(* Logix 5000 AddOnInstructionDefinition export Banner_TL50Pro_Param_v4; software revision 33.00 *)

TYPE Banner_IOL_Port_v4 :   // UDT that has all of the data items necessary to communicate with a specific Port on a IO-Link Master
STRUCT
   Port_Controlled : INT;   // Each bit represents a port on an IO-Link Master. Set to 1 to tell AOI to control that port.
   Port_Activate : INT;   // Each bit represents a port on an IO-Link Master. When ON that port will process any commands in queue.
   Port_Read : INT;   // Each bit represents a port on an IO-Link Master. Used to determine when device AOI has requested a Read command.
   Port_Write : INT;   // Each bit represents a port on an IO-Link Master. Used to determine when device AOI has requested a Write command.
   Port_RW_Complete : INT;   // Each bit represents a port on an IO-Link Master. Tells device AOI that Read or Write request has been completed.
   Port_Device_Read : INT;
   Data_Transfer : SINT[190];   // Array to transfer data from IO-Master to device AOIs.
END_STRUCT
END_TYPE

TYPE Banner_TL50Pro_Basic_SP_v4 :   // Basic parameters for a TL50 Pro segment.
STRUCT
   Animation_Rotational_Direction : SINT;   // 0 = Counter Clockwise, 1 = Clockwise
   Animation_Color_2_Intensity : SINT;   // 0 = High, 1 = Low, 2 = Medium, 3 = Off, 4 = Custom
   Animation_Color_2 : INT;   // 0 = Green, 1 = Red, 2 = Orange, 3 = Amber, 4 = Yellow, 5 = Lime Green, 6 = Spring Green, 7 = Cyan, 8 = Sky Blue, 9 = Blue, 10 = Violet, 11 = Magenta, 12 = Rose, 13 = White, 14 = Custom, 15 = Custom 2
   Animation_Pattern : SINT;   // 0 = Normal, 1 = Strobe, 2 = Three Pulse, 3 = SOS, 4 = Random
   Animation_Speed : SINT;   // 0 = Medium, 1 = Fasr, 2 = Slow, 3 = Custom
   Animation_Color_1_Intensity : SINT;   // 0 = High, 1 = Low, 2 = Medium, 3 = Off, 4 = Custom
   Animation_Color_1 : INT;   // 0 = Green, 1 = Red, 2 = Orange, 3 = Amber, 4 = Yellow, 5 = Lime Green, 6 = Spring Green, 7 = Cyan, 8 = Sky Blue, 9 = Blue, 10 = Violet, 11 = Magenta, 12 = Rose, 13 = White, 14 = Custom, 15 = Custom 2
   Animation : SINT;   // 0 = Off, 1 = Steady, 2 = Flash, 3 = Two Color, 4 = Half/Half, 5 = Half/Half Rotate, 6 = Chase, 7 = Intesnity Sweep
   Basic_Speed : SINT;   // 0 = Medium, 1 = Fast, 2 = Slow, 3 = Custom
   Basic_Color : SINT;   // 0 = Green, 1 = Red, 2 = Orange, 3 = Amber, 4 = Yellow, 5 = Lime Green, 6 = Spring Green, 7 = Cyan, 8 = Sky Blue, 9 = Blue, 10 = Violet, 11 = Magenta, 12 = Rose, 13 = White, 14 = Custom, 15 = Custom 2
END_STRUCT
END_TYPE

TYPE Banner_TL50Pro_RD_v4 :   // UDT that stores the Read Data for a TL50 Pro.
STRUCT
   Master_Cycle_Time : INT;
   Min_Cycle_Time : INT;
   M_Sequence_Capability : INT;
   IO_Link_Version_ID : INT;
   Process_Data_Input_Length : INT;
   Process_Data_Output_Length : INT;
   Combined_Vendor_ID : DINT;   // IO-Link Vendor ID
   Vendor_ID1 : INT;
   Vendor_ID2 : INT;
   Combined_Device_ID : DINT;   // IO-Link Device ID
   Device_ID1 : INT;
   Device_ID2 : INT;
   Device_ID3 : INT;
   Serial_Number : STRING;
END_STRUCT
END_TYPE

TYPE Banner_TL50Pro_v4 :   // All of the parameters for a TL50 Pro.
STRUCT
   Initial_Global_Read : BOOL;   // Determines if all of the IO-Link data has been read into the PLC yet
   Command : INT;   // Value placed in here will activate a read or write to a specifc IO-Link Index
   Read_Data : Banner_TL50Pro_RD_v4;   // Read Only Data
   Write_Data : Banner_TL50Pro_WD_v4;   // Write Data
   Archive_Data : Banner_TL50Pro_WD_v4;   // Archive of the Write Data
   Reset : BOOL;   // Resets AOI. This will force a complete parameter read of the sensor.
END_STRUCT
END_TYPE

TYPE Banner_TL50Pro_WD_v4 :   // UDT that stores the Write Data for a TL50 Pro.
STRUCT
   System_Command : INT;   // See IODD file for list of commands that can be activated via the System Command interface
   Parameter_Access_Lock : SINT;   // Write access to all parameters is prohibited while value is 1. Only this parameter can be adjusted when value is 1.
   Data_Storage_Lock : SINT;   // Automatic data storage is disabled when this value is equal to 1. Read access is not affected.
   Local_Parameterization_Lock : SINT;   // Parameterization via local control elements on device is disabled.
   Local_User_Interface_Lock : SINT;   // Operation of local user interface is disabled.
   Operating_Mode_Selection : SINT;   // 0 = Basic Mode, 1 = Advanced Mode, 2= Run Mode, 3 = Level Mode
   Segment_Basic : Banner_TL50Pro_Basic_SP_v4[11];
   Restrict_to_Gamut : SINT;   // 0 = Off, 1 = On
   Number_of_Segments_for_Scroll_and_Bounce : INT;   // 0 to 10
   Custom_Flash_Rate : INT;   // .5 to 20 Hz (range 5 to 200)
   Custom_Intensity : INT;   // 0 to 100%
   Custom_1_Red : INT;   // 0 to 255. Value of the Red portion of the RGB color value for Custom 1
   Custom_1_Green : INT;   // 0 to 255. Value of the Green portion of the RGB color value for Custom 1.
   Custom_1_Blue : INT;   // 0 to 255. Value of the Blue portion of the RGB color value for Custom 1.
   Custom_2_Red : INT;   // 0 to 255. Value of the Red portion of the RGB color value for Custom 2.
   Custom_2_Green : INT;   // 0 to 255. Value of the Green portion of the RGB color value for Custom 2.
   Custom_2_Blue : INT;   // 0 to 255. Value of the Blue portion of the RGB color value for Custom 2.
   LM_Full_Scale_Value : DINT;
   LM_Base_Color : INT;   // 0 = Green, 1 = Red, 2 = Orange, 3 = Amber, 4 = Yellow, 5 = Lime Green, 6 = Spring Green, 7 = Cyan, 8 = Sky Blue, 9 = Blue, 10 = Violet, 11 = Magenta, 12 = Rose, 13 = White, 14 = Custom, 15 = Custom 2
   LM_Base_Intensity : SINT;   // 0 = High, 1 = Low, 2 = Medium, 3 = Off, 4 = Custom
   LM_Base_State : SINT;   // 0 = Steady, 1 = Flashing
   LM_Threshold_Type : SINT;   // 0 = None, 1 = Low, 2 = High, 3 = High and Low
   LM_Low_Threshold_Value : DINT;
   LM_Low_Threshold_Color : INT;   // 0 = Green, 1 = Red, 2 = Orange, 3 = Amber, 4 = Yellow, 5 = Lime Green, 6 = Spring Green, 7 = Cyan, 8 = Sky Blue, 9 = Blue, 10 = Violet, 11 = Magenta, 12 = Rose, 13 = White, 14 = Custom, 15 = Custom 2
   LM_Low_Threshold_Intensity : SINT;   // 0 = High, 1 = Low, 2 = Medium, 3 = Off, 4 = Custom
   LM_Low_Threshold_State : SINT;   // 0 = Steady, 1 = Flashing
   LM_High_Threshold_Value : DINT;
   LM_High_Threshold_Color : INT;   // 0 = Green, 1 = Red, 2 = Orange, 3 = Amber, 4 = Yellow, 5 = Lime Green, 6 = Spring Green, 7 = Cyan, 8 = Sky Blue, 9 = Blue, 10 = Violet, 11 = Magenta, 12 = Rose, 13 = White, 14 = Custom, 15 = Custom 2
   LM_High_Threshold_Intensity : SINT;   // 0 = High, 1 = Low, 2 = Medium, 3 = Off, 4 = Custom
   LM_High_Threshold_State : SINT;   // 0 = Steady, 1 = Flashing
   LM_Flash_Rate : SINT;   // 0 = Medium, 1 = Fast, 2 = Slow, 3 = Custom
   LM_Dominance : SINT;   // 0 = Dominant, 1 = Non-Dominant
   LM_Subsegment_Style : SINT;   // 0 = Steady, 1 = Flashing, 2 = Analog
   LM_Background_Color : SINT;   // 0 = Green, 1 = Red, 2 = Orange, 3 = Amber, 4 = Yellow, 5 = Lime Green, 6 = Spring Green, 7 = Cyan, 8 = Sky Blue, 9 = Blue, 10 = Violet, 11 = Magenta, 12 = Rose, 13 = White, 14 = Custom, 15 = Custom 2
   LM_Background_Intensity : SINT;   // 0 = High, 1 = Low, 2 = Medium, 3 = Off, 4 = Custom
   LM_Orientation : SINT;   // 0 = Steady, 1 = Flashing
END_STRUCT
END_TYPE

ADD_ON_INSTRUCTION Banner_TL50Pro_Param_v4   (* revision 4.1, vendor Banner Engineering *)
// AOI to read and write parameter data to an IO-Link TL50 Pro.
VAR_IN_OUT
   TL50_Pro : Banner_TL50Pro_v4; {required}
   Port_Data : Banner_IOL_Port_v4; {required}
END_VAR
VAR_INPUT
   Port : INT; {required}   // Port Number that device is plugged into.
END_VAR
VAR
   Local_Control : DINT; {access None}
   Global_Read_Command_Value : INT; {access None}
   Global_Write_Command_Value : INT; {access None}
   Command_Being_Processed : BOOL; {access None}
   Update_Archive : BOOL; {access None}
   Index_Write_Inprocess : DINT; {access None}
   Index_Write_Control : DINT; {access None}
   Inprocess_Index : DINT; {access None}
   Index_R_Segment : DINT; {access None}
   BS_Index : DINT; {access None}
   Index_W_Segment : DINT; {access None}
   SB_W_Index : DINT; {access None}
   Index_Segment_Read : DINT; {access None}
END_VAR

ROUTINE Logic   (* ladder *)
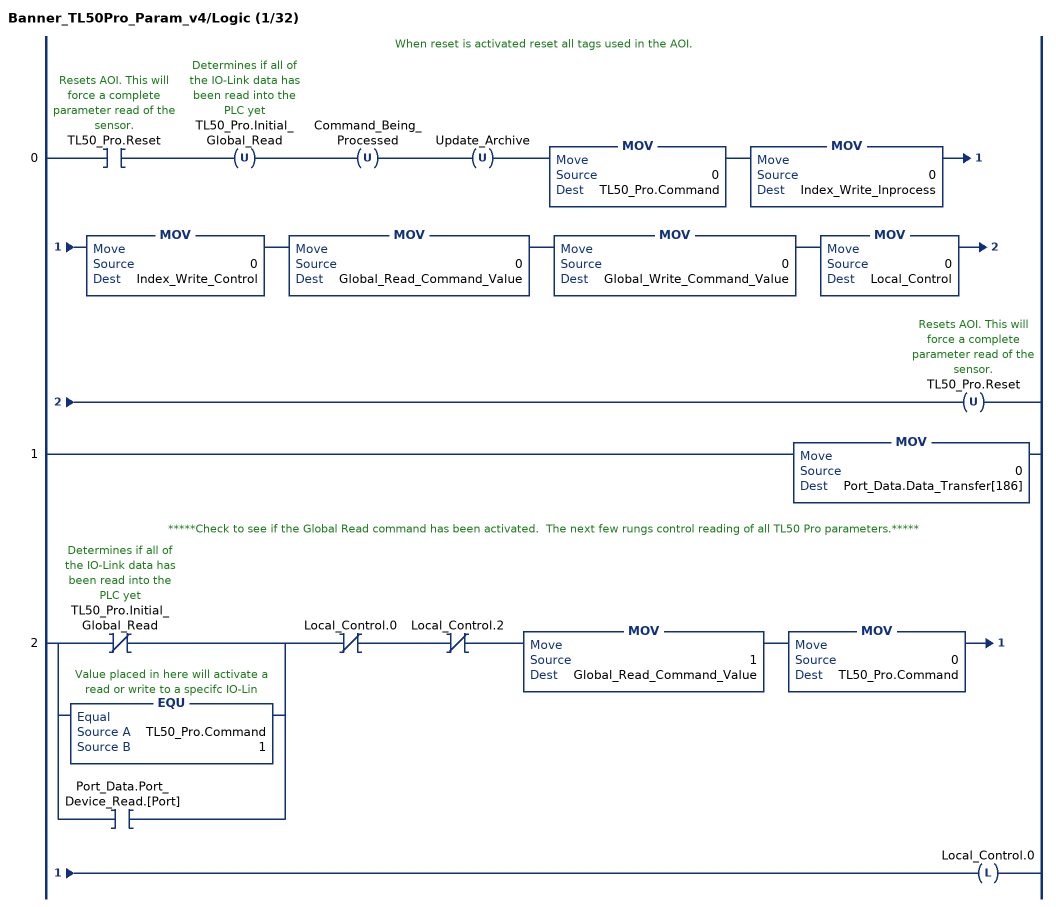
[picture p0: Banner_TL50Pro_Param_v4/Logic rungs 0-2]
   // When reset is activated reset all tags used in the AOI.
   0: XIC(TL50_Pro.Reset)OTU(TL50_Pro.Initial_Global_Read)OTU(Command_Being_Processed)OTU(Update_Archive)MOV(0,TL50_Pro.Command)MOV(0,Index_Write_Inprocess)MOV(0,Index_Write_Control)MOV(0,Global_Read_Command_Value)MOV(0,Global_Write_Command_Value)MOV(0,Local_Control)OTU(TL50_Pro.Reset);
   1: MOV(0,Port_Data.Data_Transfer[186]);
   // *****Check to see if the Global Read command has been activated.  The next few rungs control reading of all TL50 Pro parameters.*****
   2: [XIO(TL50_Pro.Initial_Global_Read) ,EQU(TL50_Pro.Command,1) ,XIC(Port_Data.Port_Device_Read.[Port]) ]XIO(Local_Control.0)XIO(Local_Control.2)MOV(1,Global_Read_Command_Value)MOV(0,TL50_Pro.Command)OTL(Local_Control.0);
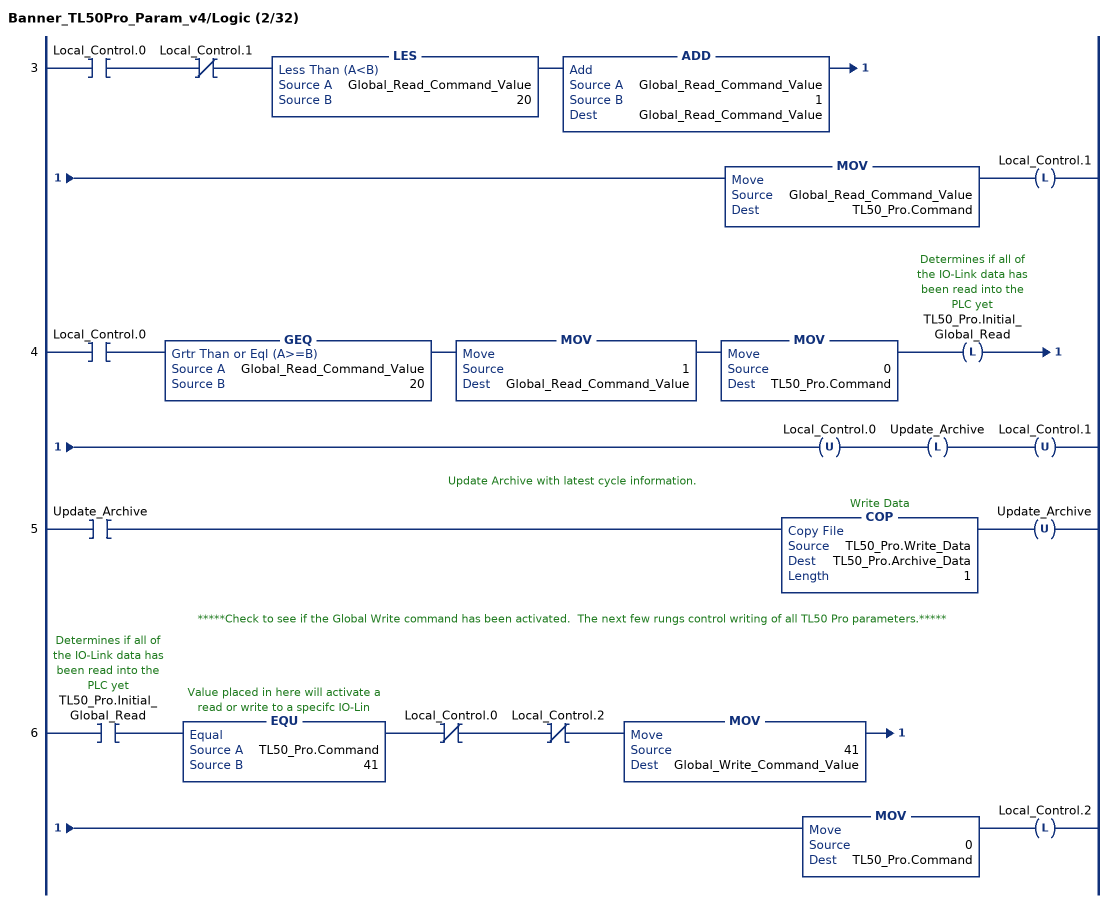
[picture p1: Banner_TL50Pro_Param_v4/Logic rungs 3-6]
   3: XIC(Local_Control.0)XIO(Local_Control.1)LES(Global_Read_Command_Value,20)ADD(Global_Read_Command_Value,1,Global_Read_Command_Value)MOV(Global_Read_Command_Value,TL50_Pro.Command)OTL(Local_Control.1);
   4: XIC(Local_Control.0)GEQ(Global_Read_Command_Value,20)MOV(1,Global_Read_Command_Value)MOV(0,TL50_Pro.Command)OTL(TL50_Pro.Initial_Global_Read)OTU(Local_Control.0)OTL(Update_Archive)OTU(Local_Control.1);
   // Update Archive with latest cycle information.
   5: XIC(Update_Archive)COP(TL50_Pro.Write_Data,TL50_Pro.Archive_Data,1)OTU(Update_Archive);
   // *****Check to see if the Global Write command has been activated.  The next few rungs control writing of all TL50 Pro parameters.*****
   6: XIC(TL50_Pro.Initial_Global_Read)EQU(TL50_Pro.Command,41)XIO(Local_Control.0)XIO(Local_Control.2)MOV(41,Global_Write_Command_Value)MOV(0,TL50_Pro.Command)OTL(Local_Control.2);
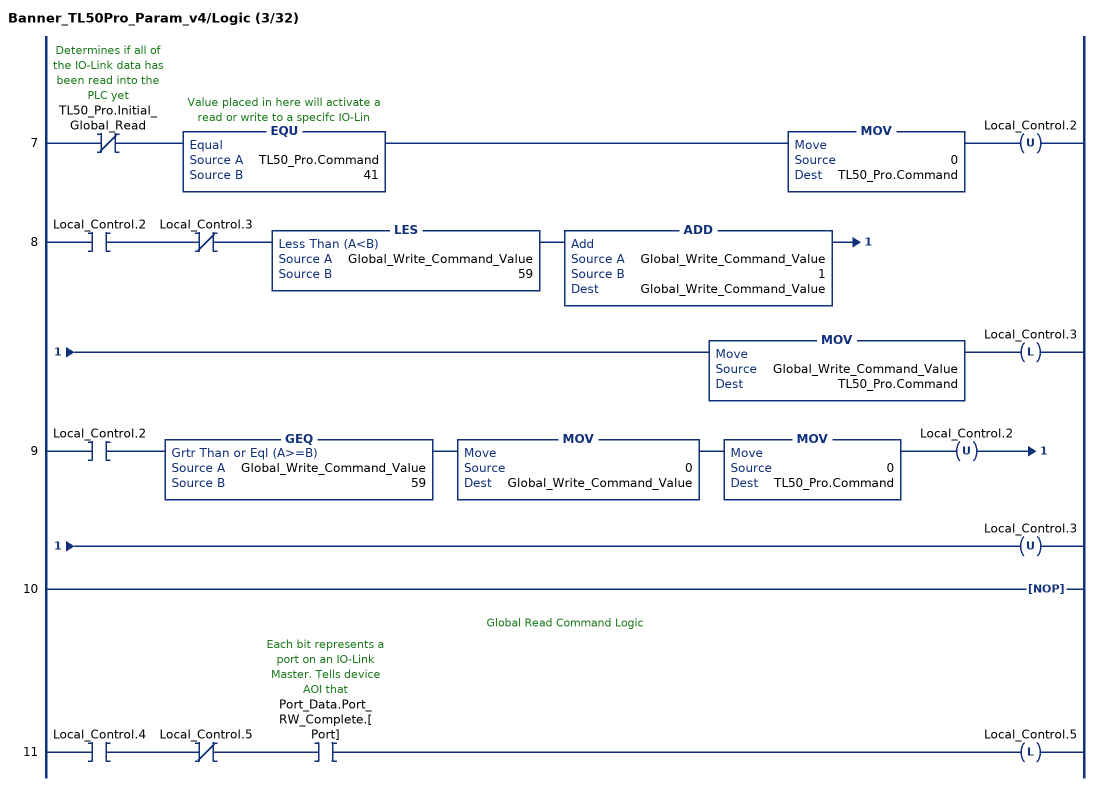
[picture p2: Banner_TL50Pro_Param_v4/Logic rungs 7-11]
   7: XIO(TL50_Pro.Initial_Global_Read)EQU(TL50_Pro.Command,41)MOV(0,TL50_Pro.Command)OTU(Local_Control.2);
   8: XIC(Local_Control.2)XIO(Local_Control.3)LES(Global_Write_Command_Value,59)ADD(Global_Write_Command_Value,1,Global_Write_Command_Value)MOV(Global_Write_Command_Value,TL50_Pro.Command)OTL(Local_Control.3);
   9: XIC(Local_Control.2)GEQ(Global_Write_Command_Value,59)MOV(0,Global_Write_Command_Value)MOV(0,TL50_Pro.Command)OTU(Local_Control.2)OTU(Local_Control.3);
   10: NOP();
   // Global Read Command Logic
   11: XIC(Local_Control.4)XIO(Local_Control.5)XIC(Port_Data.Port_RW_Complete.[Port])OTL(Local_Control.5);
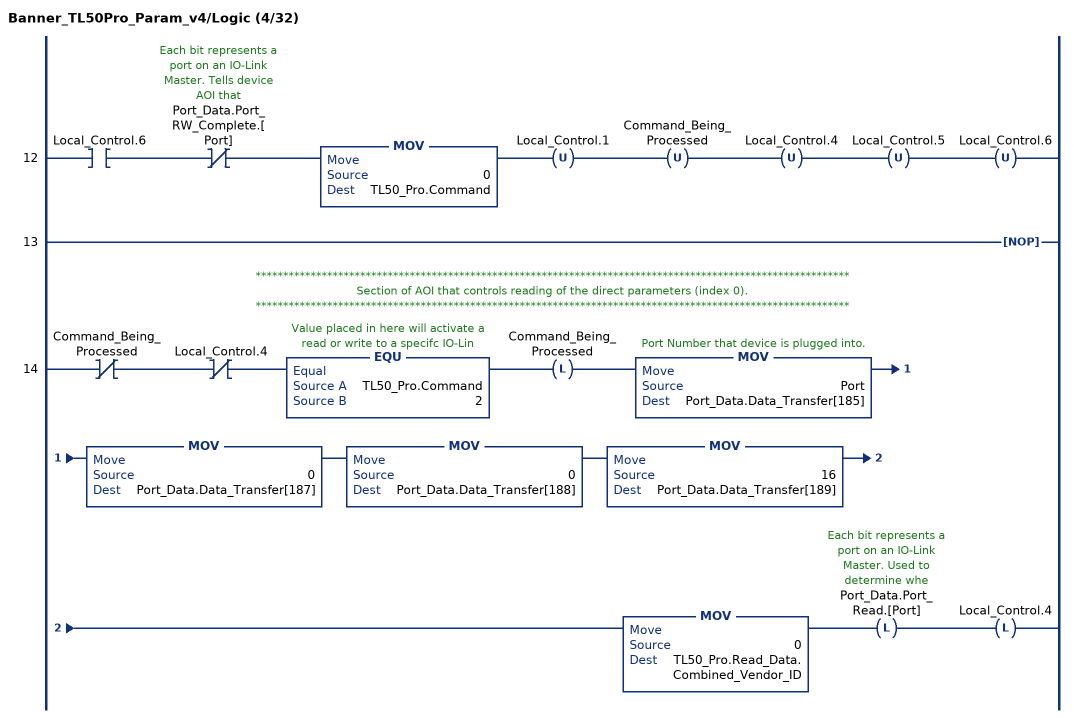
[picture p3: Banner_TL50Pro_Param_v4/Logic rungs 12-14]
   12: XIC(Local_Control.6)XIO(Port_Data.Port_RW_Complete.[Port])MOV(0,TL50_Pro.Command)OTU(Local_Control.1)OTU(Command_Being_Processed)OTU(Local_Control.4)OTU(Local_Control.5)OTU(Local_Control.6);
   13: NOP();
   // ************************************************************************************************************
   // Section of AOI that controls reading of the direct parameters (index 0).
   // ************************************************************************************************************
   14: XIO(Command_Being_Processed)XIO(Local_Control.4)EQU(TL50_Pro.Command,2)OTL(Command_Being_Processed)MOV(Port,Port_Data.Data_Transfer[185])MOV(0,Port_Data.Data_Transfer[187])MOV(0,Port_Data.Data_Transfer[188])MOV(16,Port_Data.Data_Transfer[189])MOV(0,TL50_Pro.Read_Data.Combined_Vendor_ID)OTL(Port_Data.Port_Read.[Port])OTL(Local_Control.4);
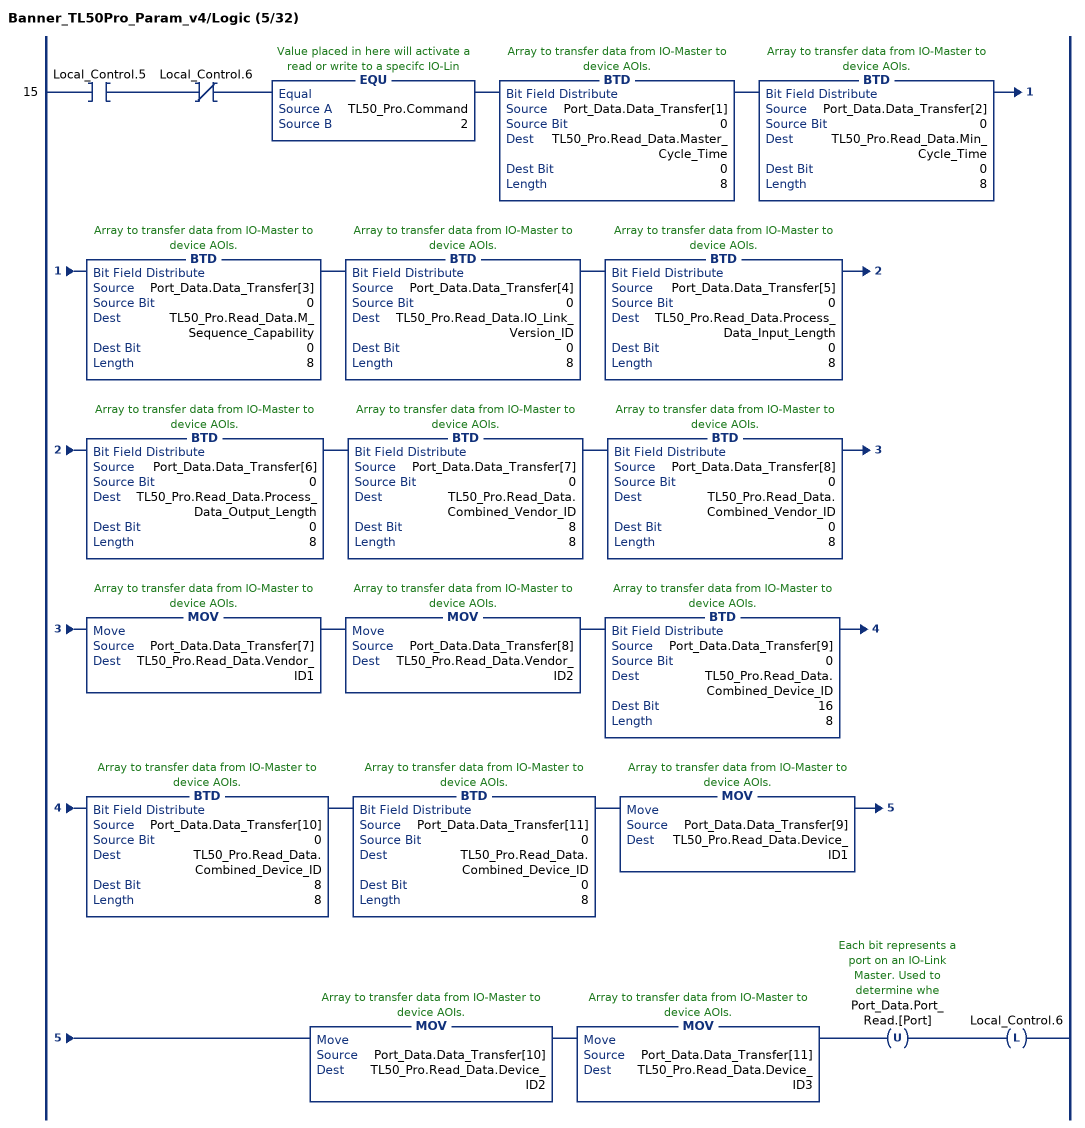
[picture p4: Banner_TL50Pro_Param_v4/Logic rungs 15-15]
   15: XIC(Local_Control.5)XIO(Local_Control.6)EQU(TL50_Pro.Command,2)BTD(Port_Data.Data_Transfer[1],0,TL50_Pro.Read_Data.Master_Cycle_Time,0,8)BTD(Port_Data.Data_Transfer[2],0,TL50_Pro.Read_Data.Min_Cycle_Time,0,8)BTD(Port_Data.Data_Transfer[3],0,TL50_Pro.Read_Data.M_Sequence_Capability,0,8)BTD(Port_Data.Data_Transfer[4],0,TL50_Pro.Read_Data.IO_Link_Version_ID,0,8)BTD(Port_Data.Data_Transfer[5],0,TL50_Pro.Read_Data.Process_Data_Input_Length,0,8)BTD(Port_Data.Data_Transfer[6],0,TL50_Pro.Read_Data.Process_Data_Output_Length,0,8)BTD(Port_Data.Data_Transfer[7],0,TL50_Pro.Read_Data.Combined_Vendor_ID,8,8)BTD(Port_Data.Data_Transfer[8],0,TL50_Pro.Read_Data.Combined_Vendor_ID,0,8)MOV(Port_Data.Data_Transfer[7],TL50_Pro.Read_Data.Vendor_ID1)MOV(Port_Data.Data_Transfer[8],TL50_Pro.Read_Data.Vendor_ID2)BTD(Port_Data.Data_Transfer[9],0,TL50_Pro.Read_Data.Combined_Device_ID,16,8)BTD(Port_Data.Data_Transfer[10],0,TL50_Pro.Read_Data.Combined_Device_ID,8,8)BTD(Port_Data.Data_Transfer[11],0,TL50_Pro.Read_Data.Combined_Device_ID,0,8)MOV(Port_Data.Data_Transfer[9],TL50_Pro.Read_Data.Device_ID1)MOV(Port_Data.Data_Transfer[10],TL50_Pro.Read_Data.Device_ID2)MOV(Port_Data.Data_Transfer[11],TL50_Pro.Read_Data.Device_ID3)OTU(Port_Data.Port_Read.[Port])OTL(Local_Control.6);
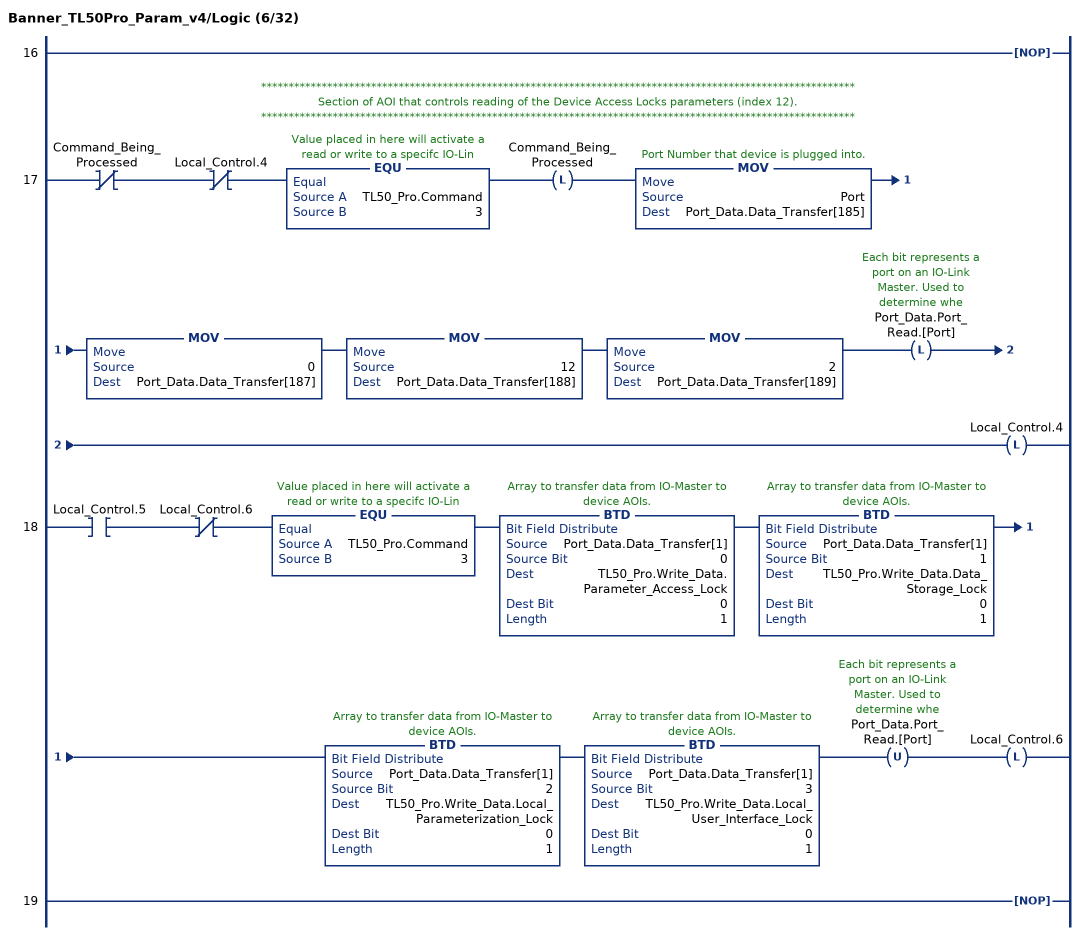
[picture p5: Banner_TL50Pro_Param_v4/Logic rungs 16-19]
   16: NOP();
   // ************************************************************************************************************
   // Section of AOI that controls reading of the Device Access Locks parameters (index 12).
   // ************************************************************************************************************
   17: XIO(Command_Being_Processed)XIO(Local_Control.4)EQU(TL50_Pro.Command,3)OTL(Command_Being_Processed)MOV(Port,Port_Data.Data_Transfer[185])MOV(0,Port_Data.Data_Transfer[187])MOV(12,Port_Data.Data_Transfer[188])MOV(2,Port_Data.Data_Transfer[189])OTL(Port_Data.Port_Read.[Port])OTL(Local_Control.4);
   18: XIC(Local_Control.5)XIO(Local_Control.6)EQU(TL50_Pro.Command,3)BTD(Port_Data.Data_Transfer[1],0,TL50_Pro.Write_Data.Parameter_Access_Lock,0,1)BTD(Port_Data.Data_Transfer[1],1,TL50_Pro.Write_Data.Data_Storage_Lock,0,1)BTD(Port_Data.Data_Transfer[1],2,TL50_Pro.Write_Data.Local_Parameterization_Lock,0,1)BTD(Port_Data.Data_Transfer[1],3,TL50_Pro.Write_Data.Local_User_Interface_Lock,0,1)OTU(Port_Data.Port_Read.[Port])OTL(Local_Control.6);
   19: NOP();
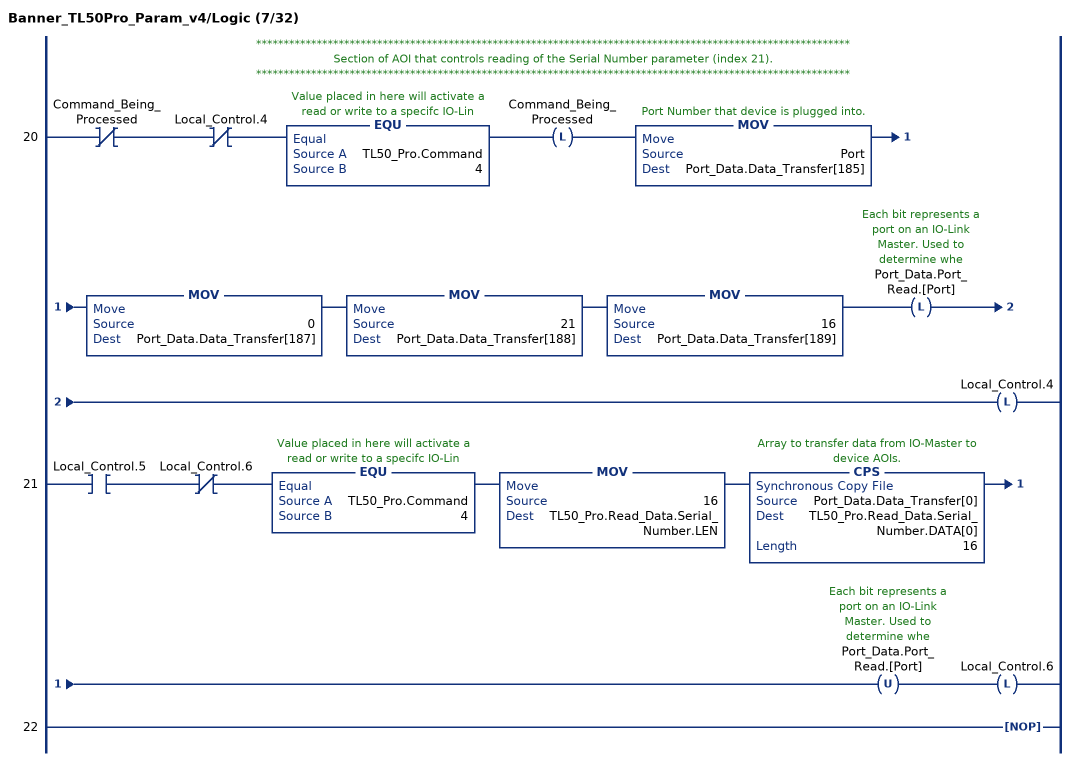
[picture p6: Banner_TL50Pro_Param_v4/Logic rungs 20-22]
   // ************************************************************************************************************
   // Section of AOI that controls reading of the Serial Number parameter (index 21).
   // ************************************************************************************************************
   20: XIO(Command_Being_Processed)XIO(Local_Control.4)EQU(TL50_Pro.Command,4)OTL(Command_Being_Processed)MOV(Port,Port_Data.Data_Transfer[185])MOV(0,Port_Data.Data_Transfer[187])MOV(21,Port_Data.Data_Transfer[188])MOV(16,Port_Data.Data_Transfer[189])OTL(Port_Data.Port_Read.[Port])OTL(Local_Control.4);
   21: XIC(Local_Control.5)XIO(Local_Control.6)EQU(TL50_Pro.Command,4)MOV(16,TL50_Pro.Read_Data.Serial_Number.LEN)CPS(Port_Data.Data_Transfer[0],TL50_Pro.Read_Data.Serial_Number.DATA[0],16)OTU(Port_Data.Port_Read.[Port])OTL(Local_Control.6);
   22: NOP();
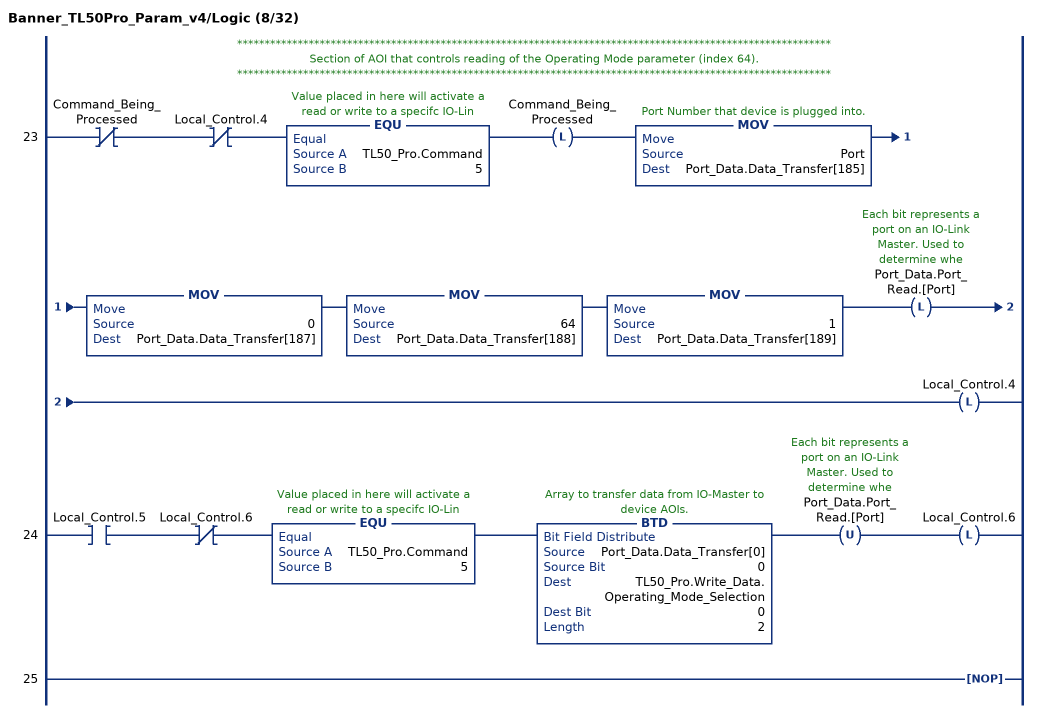
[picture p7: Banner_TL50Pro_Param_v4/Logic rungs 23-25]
   // ************************************************************************************************************
   // Section of AOI that controls reading of the Operating Mode parameter (index 64).
   // ************************************************************************************************************
   23: XIO(Command_Being_Processed)XIO(Local_Control.4)EQU(TL50_Pro.Command,5)OTL(Command_Being_Processed)MOV(Port,Port_Data.Data_Transfer[185])MOV(0,Port_Data.Data_Transfer[187])MOV(64,Port_Data.Data_Transfer[188])MOV(1,Port_Data.Data_Transfer[189])OTL(Port_Data.Port_Read.[Port])OTL(Local_Control.4);
   24: XIC(Local_Control.5)XIO(Local_Control.6)EQU(TL50_Pro.Command,5)BTD(Port_Data.Data_Transfer[0],0,TL50_Pro.Write_Data.Operating_Mode_Selection,0,2)OTU(Port_Data.Port_Read.[Port])OTL(Local_Control.6);
   25: NOP();
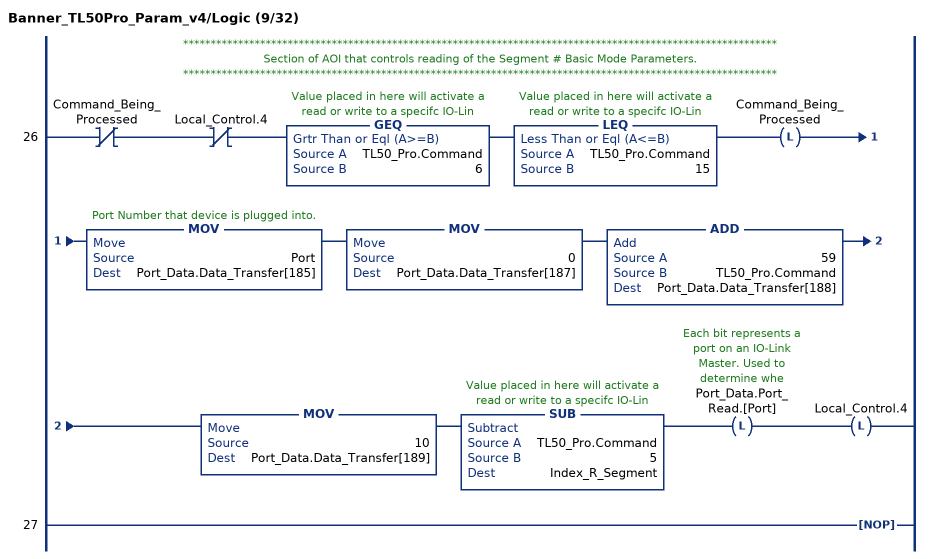
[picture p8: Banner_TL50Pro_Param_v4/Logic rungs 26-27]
   // ************************************************************************************************************
   // Section of AOI that controls reading of the Segment # Basic Mode Parameters.
   // ************************************************************************************************************
   26: XIO(Command_Being_Processed)XIO(Local_Control.4)GEQ(TL50_Pro.Command,6)LEQ(TL50_Pro.Command,15)OTL(Command_Being_Processed)MOV(Port,Port_Data.Data_Transfer[185])MOV(0,Port_Data.Data_Transfer[187])ADD(59,TL50_Pro.Command,Port_Data.Data_Transfer[188])MOV(10,Port_Data.Data_Transfer[189])SUB(TL50_Pro.Command,5,Index_R_Segment)OTL(Port_Data.Port_Read.[Port])OTL(Local_Control.4);
   27: NOP();
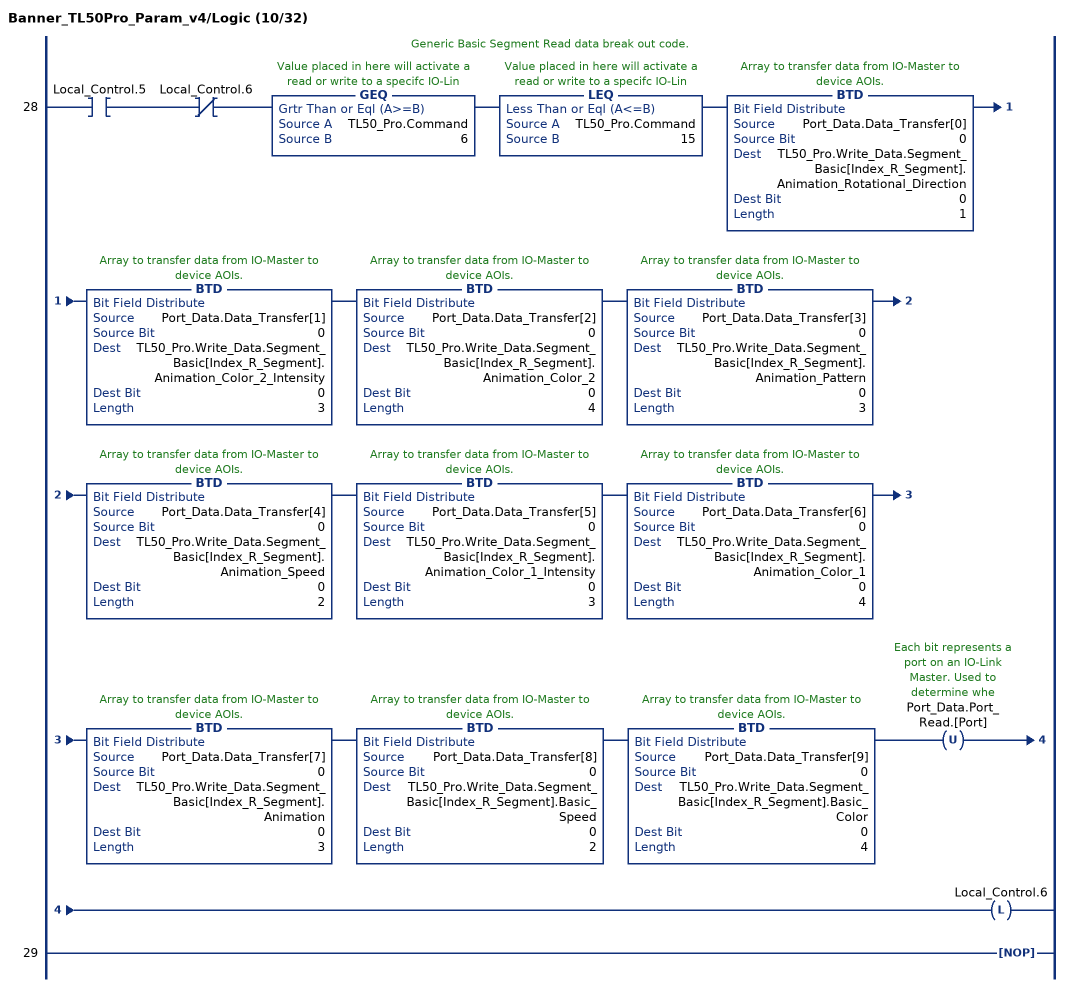
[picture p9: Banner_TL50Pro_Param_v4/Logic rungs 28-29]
   // Generic Basic Segment Read data break out code.
   28: XIC(Local_Control.5)XIO(Local_Control.6)GEQ(TL50_Pro.Command,6)LEQ(TL50_Pro.Command,15)BTD(Port_Data.Data_Transfer[0],0,TL50_Pro.Write_Data.Segment_Basic[Index_R_Segment].Animation_Rotational_Direction,0,1)BTD(Port_Data.Data_Transfer[1],0,TL50_Pro.Write_Data.Segment_Basic[Index_R_Segment].Animation_Color_2_Intensity,0,3)BTD(Port_Data.Data_Transfer[2],0,TL50_Pro.Write_Data.Segment_Basic[Index_R_Segment].Animation_Color_2,0,4)BTD(Port_Data.Data_Transfer[3],0,TL50_Pro.Write_Data.Segment_Basic[Index_R_Segment].Animation_Pattern,0,3)BTD(Port_Data.Data_Transfer[4],0,TL50_Pro.Write_Data.Segment_Basic[Index_R_Segment].Animation_Speed,0,2)BTD(Port_Data.Data_Transfer[5],0,TL50_Pro.Write_Data.Segment_Basic[Index_R_Segment].Animation_Color_1_Intensity,0,3)BTD(Port_Data.Data_Transfer[6],0,TL50_Pro.Write_Data.Segment_Basic[Index_R_Segment].Animation_Color_1,0,4)BTD(Port_Data.Data_Transfer[7],0,TL50_Pro.Write_Data.Segment_Basic[Index_R_Segment].Animation,0,3)BTD(Port_Data.Data_Transfer[8],0,TL50_Pro.Write_Data.Segment_Basic[Index_R_Segment].Basic_Speed,0,2)BTD(Port_Data.Data_Transfer[9],0,TL50_Pro.Write_Data.Segment_Basic[Index_R_Segment].Basic_Color,0,4)OTU(Port_Data.Port_Read.[Port])OTL(Local_Control.6);
   29: NOP();
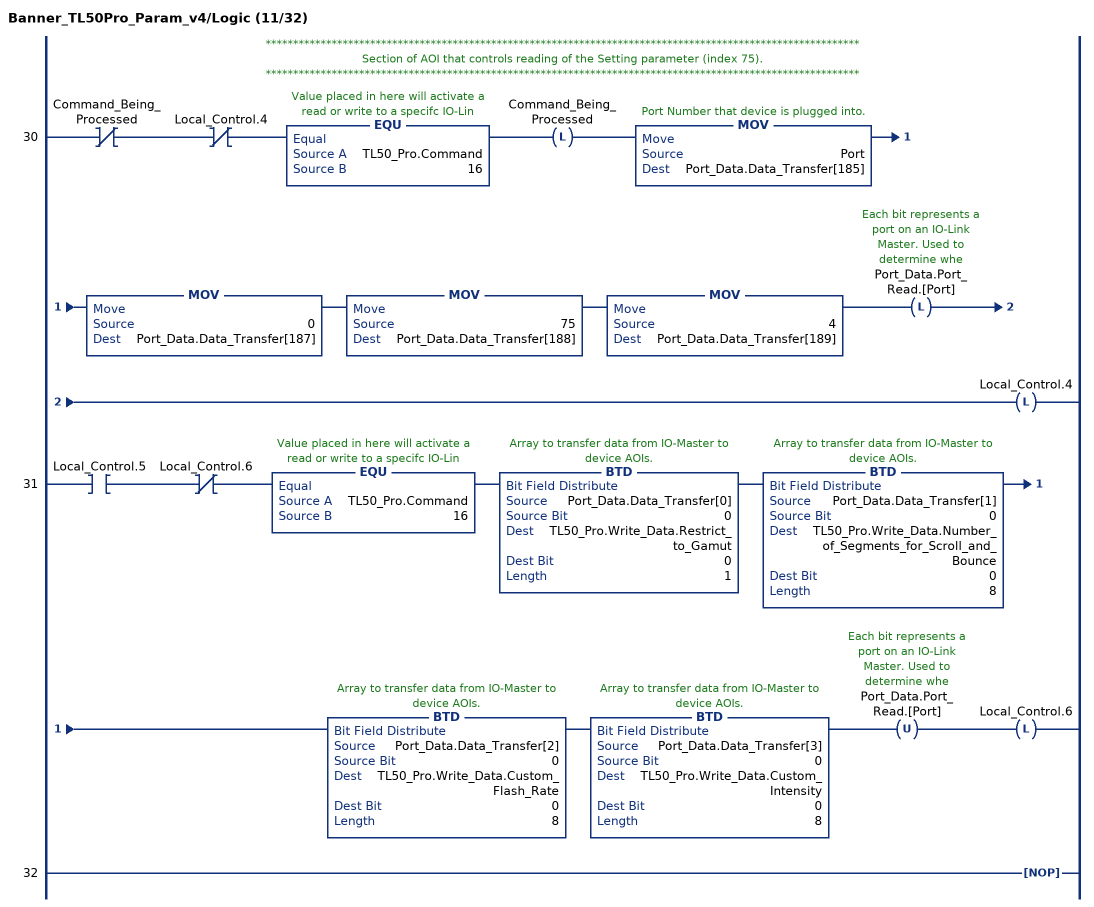
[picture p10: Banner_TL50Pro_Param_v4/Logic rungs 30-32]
   // ************************************************************************************************************
   // Section of AOI that controls reading of the Setting parameter (index 75).
   // ************************************************************************************************************
   30: XIO(Command_Being_Processed)XIO(Local_Control.4)EQU(TL50_Pro.Command,16)OTL(Command_Being_Processed)MOV(Port,Port_Data.Data_Transfer[185])MOV(0,Port_Data.Data_Transfer[187])MOV(75,Port_Data.Data_Transfer[188])MOV(4,Port_Data.Data_Transfer[189])OTL(Port_Data.Port_Read.[Port])OTL(Local_Control.4);
   31: XIC(Local_Control.5)XIO(Local_Control.6)EQU(TL50_Pro.Command,16)BTD(Port_Data.Data_Transfer[0],0,TL50_Pro.Write_Data.Restrict_to_Gamut,0,1)BTD(Port_Data.Data_Transfer[1],0,TL50_Pro.Write_Data.Number_of_Segments_for_Scroll_and_Bounce,0,8)BTD(Port_Data.Data_Transfer[2],0,TL50_Pro.Write_Data.Custom_Flash_Rate,0,8)BTD(Port_Data.Data_Transfer[3],0,TL50_Pro.Write_Data.Custom_Intensity,0,8)OTU(Port_Data.Port_Read.[Port])OTL(Local_Control.6);
   32: NOP();
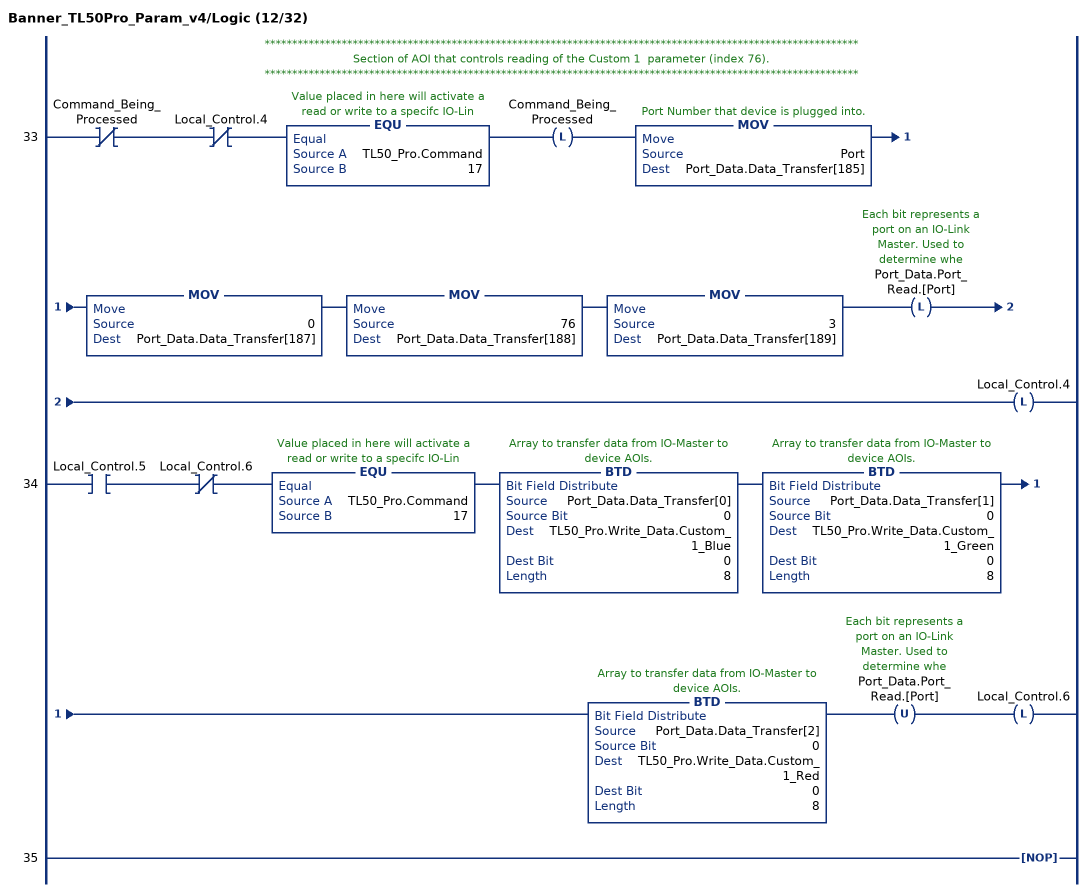
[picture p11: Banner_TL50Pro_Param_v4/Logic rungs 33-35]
   // ************************************************************************************************************
   // Section of AOI that controls reading of the Custom 1  parameter (index 76).
   // ************************************************************************************************************
   33: XIO(Command_Being_Processed)XIO(Local_Control.4)EQU(TL50_Pro.Command,17)OTL(Command_Being_Processed)MOV(Port,Port_Data.Data_Transfer[185])MOV(0,Port_Data.Data_Transfer[187])MOV(76,Port_Data.Data_Transfer[188])MOV(3,Port_Data.Data_Transfer[189])OTL(Port_Data.Port_Read.[Port])OTL(Local_Control.4);
   34: XIC(Local_Control.5)XIO(Local_Control.6)EQU(TL50_Pro.Command,17)BTD(Port_Data.Data_Transfer[0],0,TL50_Pro.Write_Data.Custom_1_Blue,0,8)BTD(Port_Data.Data_Transfer[1],0,TL50_Pro.Write_Data.Custom_1_Green,0,8)BTD(Port_Data.Data_Transfer[2],0,TL50_Pro.Write_Data.Custom_1_Red,0,8)OTU(Port_Data.Port_Read.[Port])OTL(Local_Control.6);
   35: NOP();
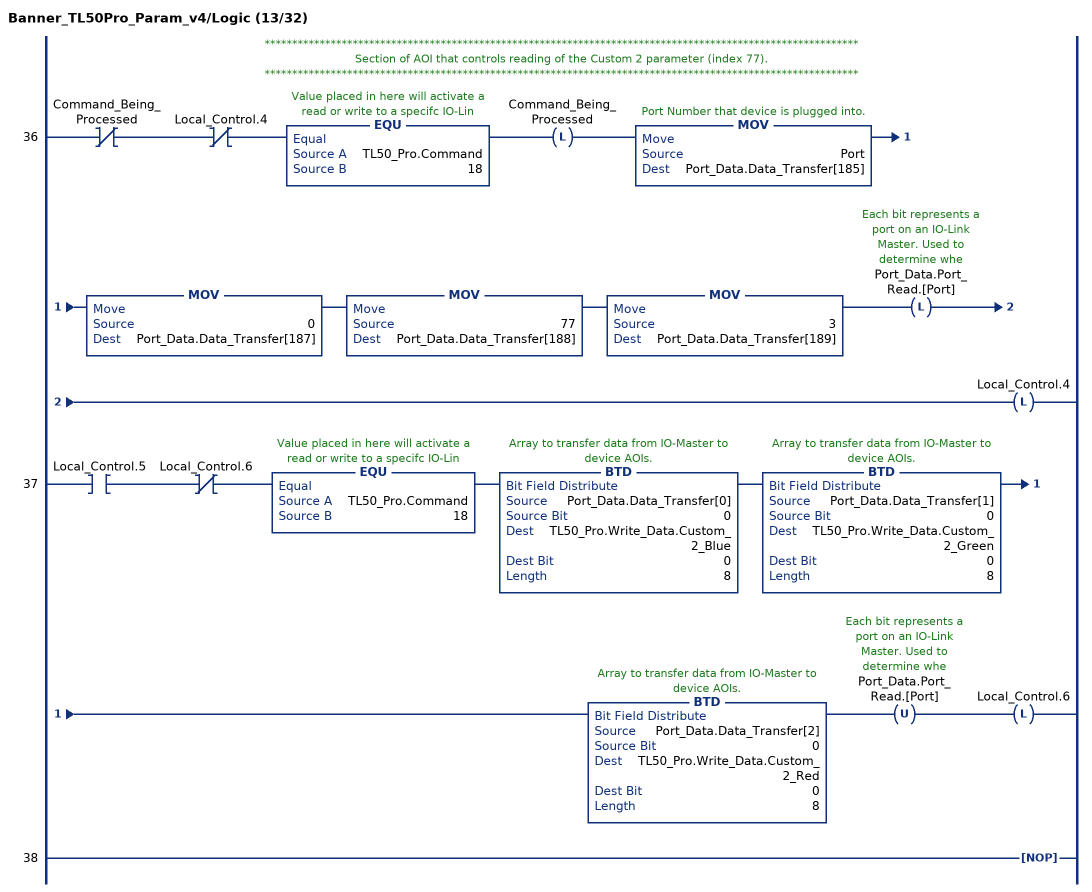
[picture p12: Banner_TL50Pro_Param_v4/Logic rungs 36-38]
   // ************************************************************************************************************
   // Section of AOI that controls reading of the Custom 2 parameter (index 77).
   // ************************************************************************************************************
   36: XIO(Command_Being_Processed)XIO(Local_Control.4)EQU(TL50_Pro.Command,18)OTL(Command_Being_Processed)MOV(Port,Port_Data.Data_Transfer[185])MOV(0,Port_Data.Data_Transfer[187])MOV(77,Port_Data.Data_Transfer[188])MOV(3,Port_Data.Data_Transfer[189])OTL(Port_Data.Port_Read.[Port])OTL(Local_Control.4);
   37: XIC(Local_Control.5)XIO(Local_Control.6)EQU(TL50_Pro.Command,18)BTD(Port_Data.Data_Transfer[0],0,TL50_Pro.Write_Data.Custom_2_Blue,0,8)BTD(Port_Data.Data_Transfer[1],0,TL50_Pro.Write_Data.Custom_2_Green,0,8)BTD(Port_Data.Data_Transfer[2],0,TL50_Pro.Write_Data.Custom_2_Red,0,8)OTU(Port_Data.Port_Read.[Port])OTL(Local_Control.6);
   38: NOP();
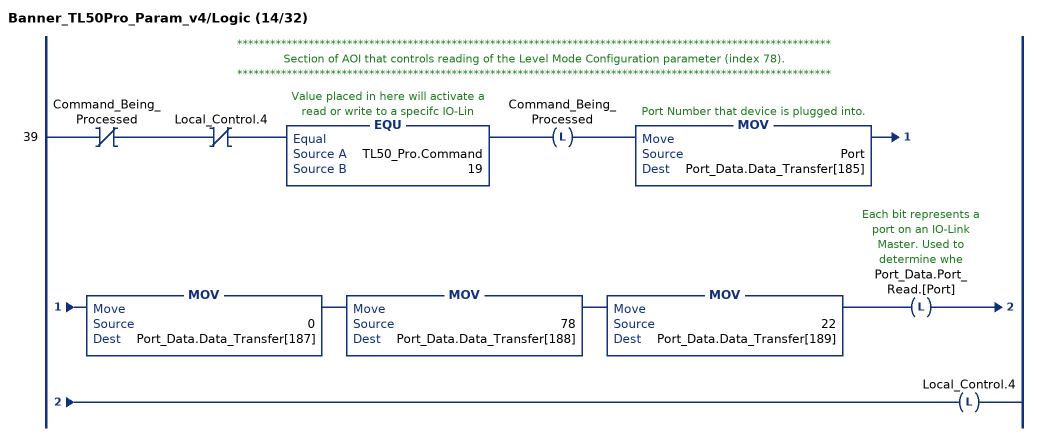
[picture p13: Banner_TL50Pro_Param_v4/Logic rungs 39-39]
   // ************************************************************************************************************
   // Section of AOI that controls reading of the Level Mode Configuration parameter (index 78).
   // ************************************************************************************************************
   39: XIO(Command_Being_Processed)XIO(Local_Control.4)EQU(TL50_Pro.Command,19)OTL(Command_Being_Processed)MOV(Port,Port_Data.Data_Transfer[185])MOV(0,Port_Data.Data_Transfer[187])MOV(78,Port_Data.Data_Transfer[188])MOV(22,Port_Data.Data_Transfer[189])OTL(Port_Data.Port_Read.[Port])OTL(Local_Control.4);
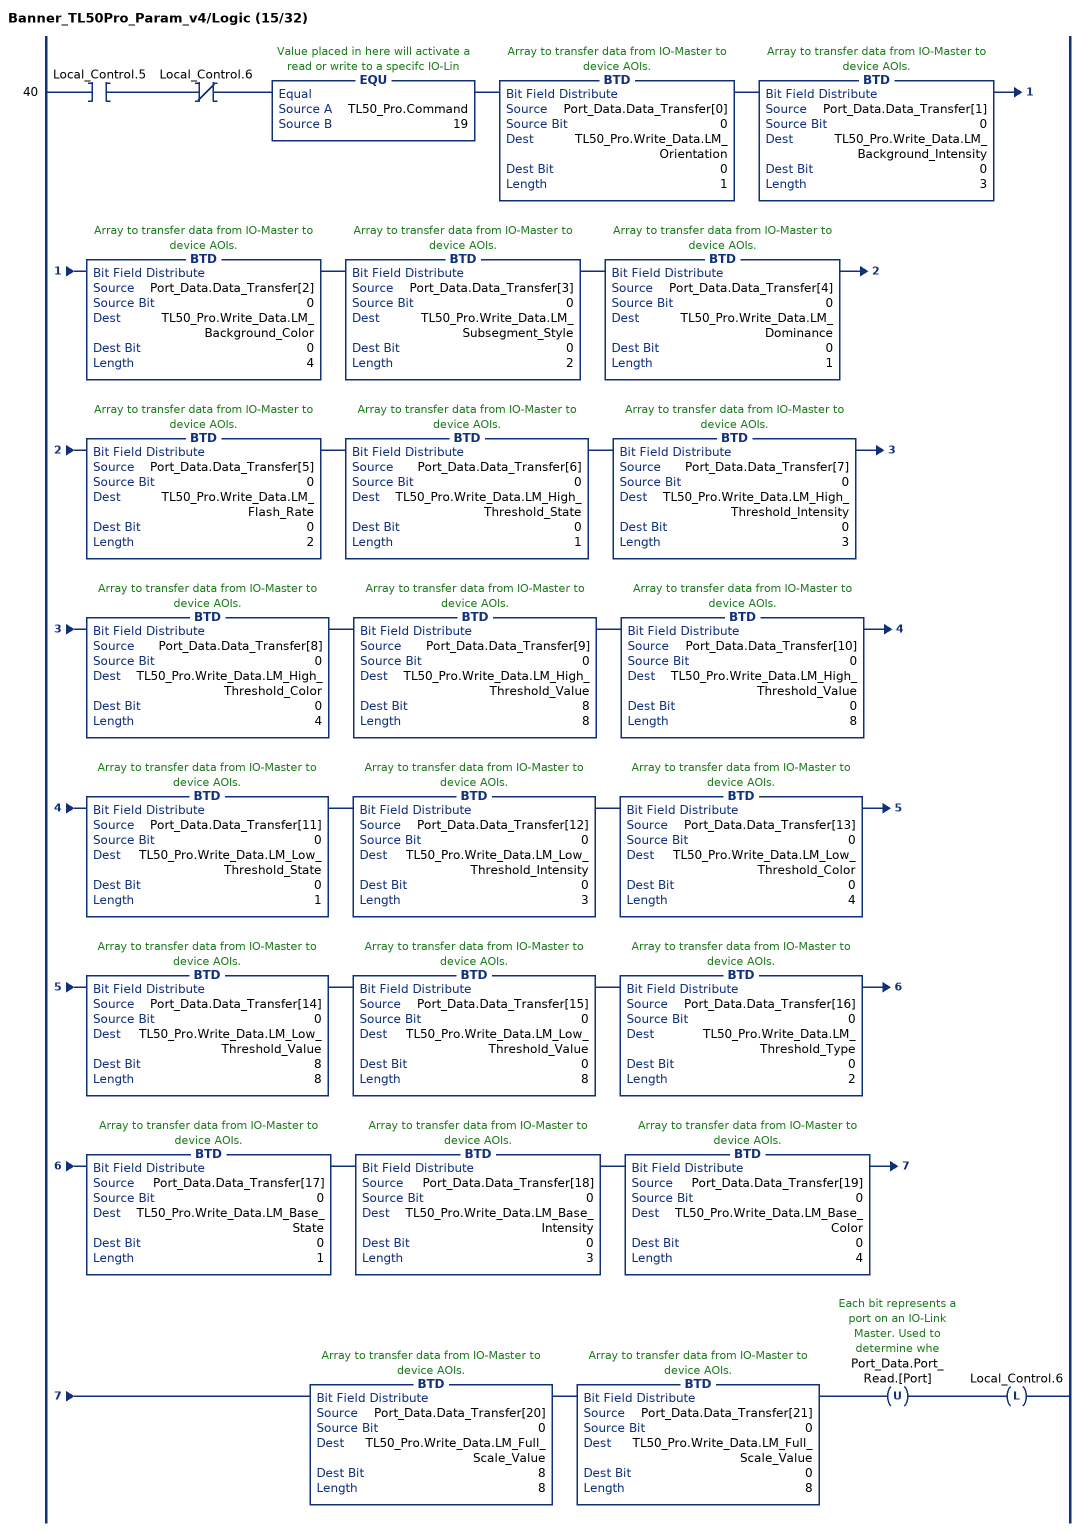
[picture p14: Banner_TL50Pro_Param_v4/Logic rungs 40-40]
   40: XIC(Local_Control.5)XIO(Local_Control.6)EQU(TL50_Pro.Command,19)BTD(Port_Data.Data_Transfer[0],0,TL50_Pro.Write_Data.LM_Orientation,0,1)BTD(Port_Data.Data_Transfer[1],0,TL50_Pro.Write_Data.LM_Background_Intensity,0,3)BTD(Port_Data.Data_Transfer[2],0,TL50_Pro.Write_Data.LM_Background_Color,0,4)BTD(Port_Data.Data_Transfer[3],0,TL50_Pro.Write_Data.LM_Subsegment_Style,0,2)BTD(Port_Data.Data_Transfer[4],0,TL50_Pro.Write_Data.LM_Dominance,0,1)BTD(Port_Data.Data_Transfer[5],0,TL50_Pro.Write_Data.LM_Flash_Rate,0,2)BTD(Port_Data.Data_Transfer[6],0,TL50_Pro.Write_Data.LM_High_Threshold_State,0,1)BTD(Port_Data.Data_Transfer[7],0,TL50_Pro.Write_Data.LM_High_Threshold_Intensity,0,3)BTD(Port_Data.Data_Transfer[8],0,TL50_Pro.Write_Data.LM_High_Threshold_Color,0,4)BTD(Port_Data.Data_Transfer[9],0,TL50_Pro.Write_Data.LM_High_Threshold_Value,8,8)BTD(Port_Data.Data_Transfer[10],0,TL50_Pro.Write_Data.LM_High_Threshold_Value,0,8)BTD(Port_Data.Data_Transfer[11],0,TL50_Pro.Write_Data.LM_Low_Threshold_State,0,1)BTD(Port_Data.Data_Transfer[12],0,TL50_Pro.Write_Data.LM_Low_Threshold_Intensity,0,3)BTD(Port_Data.Data_Transfer[13],0,TL50_Pro.Write_Data.LM_Low_Threshold_Color,0,4)BTD(Port_Data.Data_Transfer[14],0,TL50_Pro.Write_Data.LM_Low_Threshold_Value,8,8)BTD(Port_Data.Data_Transfer[15],0,TL50_Pro.Write_Data.LM_Low_Threshold_Value,0,8)BTD(Port_Data.Data_Transfer[16],0,TL50_Pro.Write_Data.LM_Threshold_Type,0,2)BTD(Port_Data.Data_Transfer[17],0,TL50_Pro.Write_Data.LM_Base_State,0,1)BTD(Port_Data.Data_Transfer[18],0,TL50_Pro.Write_Data.LM_Base_Intensity,0,3)BTD(Port_Data.Data_Transfer[19],0,TL50_Pro.Write_Data.LM_Base_Color,0,4)BTD(Port_Data.Data_Transfer[20],0,TL50_Pro.Write_Data.LM_Full_Scale_Value,8,8)BTD(Port_Data.Data_Transfer[21],0,TL50_Pro.Write_Data.LM_Full_Scale_Value,0,8)OTU(Port_Data.Port_Read.[Port])OTL(Local_Control.6);
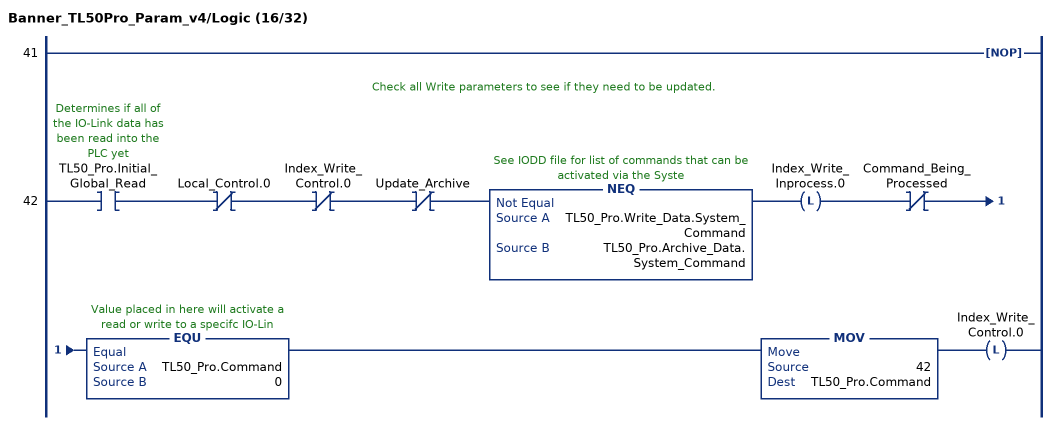
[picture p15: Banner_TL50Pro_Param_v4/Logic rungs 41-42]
   41: NOP();
   // Check all Write parameters to see if they need to be updated.
   42: XIC(TL50_Pro.Initial_Global_Read)XIO(Local_Control.0)XIO(Index_Write_Control.0)XIO(Update_Archive)NEQ(TL50_Pro.Write_Data.System_Command,TL50_Pro.Archive_Data.System_Command)OTL(Index_Write_Inprocess.0)XIO(Command_Being_Processed)EQU(TL50_Pro.Command,0)MOV(42,TL50_Pro.Command)OTL(Index_Write_Control.0);
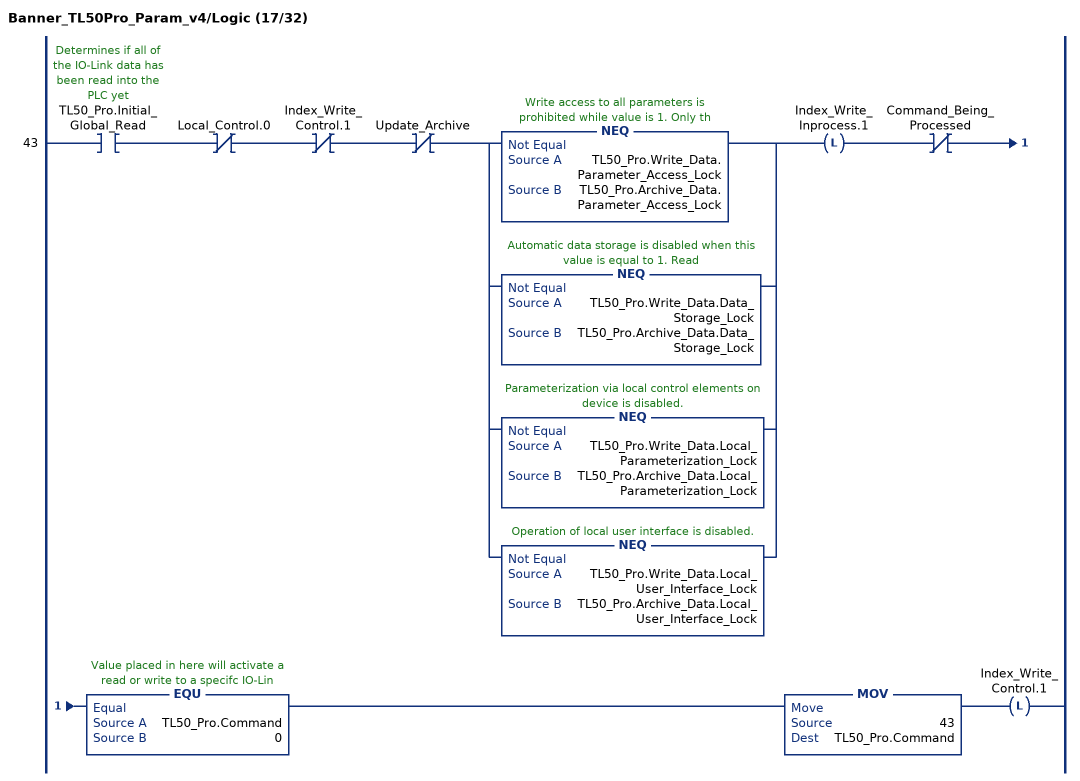
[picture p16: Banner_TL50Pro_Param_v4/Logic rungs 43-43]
   43: XIC(TL50_Pro.Initial_Global_Read)XIO(Local_Control.0)XIO(Index_Write_Control.1)XIO(Update_Archive)[NEQ(TL50_Pro.Write_Data.Parameter_Access_Lock,TL50_Pro.Archive_Data.Parameter_Access_Lock) ,NEQ(TL50_Pro.Write_Data.Data_Storage_Lock,TL50_Pro.Archive_Data.Data_Storage_Lock) ,NEQ(TL50_Pro.Write_Data.Local_Parameterization_Lock,TL50_Pro.Archive_Data.Local_Parameterization_Lock) ,NEQ(TL50_Pro.Write_Data.Local_User_Interface_Lock,TL50_Pro.Archive_Data.Local_User_Interface_Lock) ]OTL(Index_Write_Inprocess.1)XIO(Command_Being_Processed)EQU(TL50_Pro.Command,0)MOV(43,TL50_Pro.Command)OTL(Index_Write_Control.1);
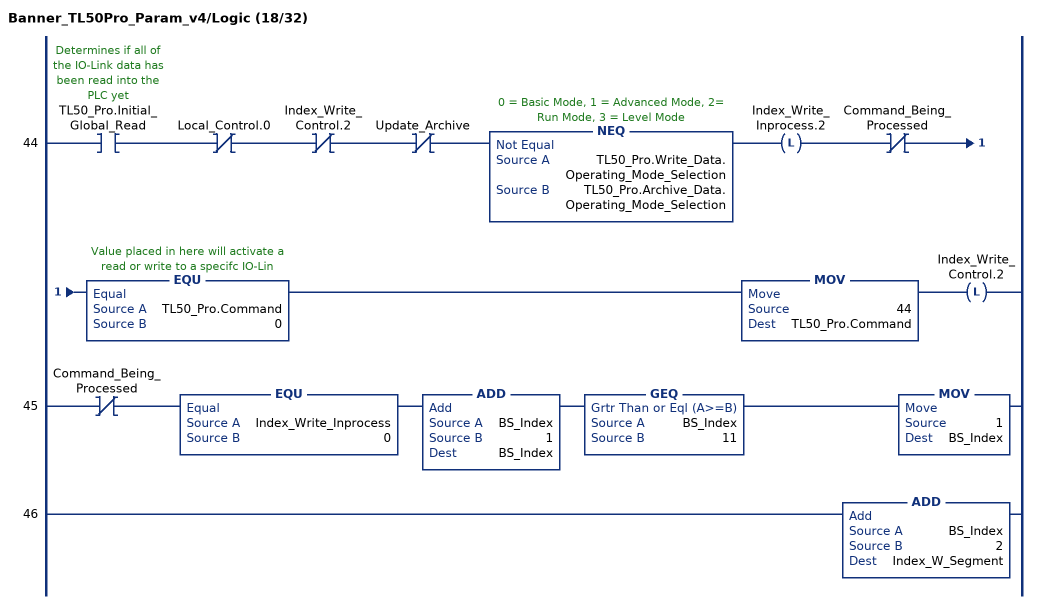
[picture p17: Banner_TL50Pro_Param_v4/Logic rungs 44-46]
   44: XIC(TL50_Pro.Initial_Global_Read)XIO(Local_Control.0)XIO(Index_Write_Control.2)XIO(Update_Archive)NEQ(TL50_Pro.Write_Data.Operating_Mode_Selection,TL50_Pro.Archive_Data.Operating_Mode_Selection)OTL(Index_Write_Inprocess.2)XIO(Command_Being_Processed)EQU(TL50_Pro.Command,0)MOV(44,TL50_Pro.Command)OTL(Index_Write_Control.2);
   45: XIO(Command_Being_Processed)EQU(Index_Write_Inprocess,0)ADD(BS_Index,1,BS_Index)GEQ(BS_Index,11)MOV(1,BS_Index);
   46: ADD(BS_Index,2,Index_W_Segment);
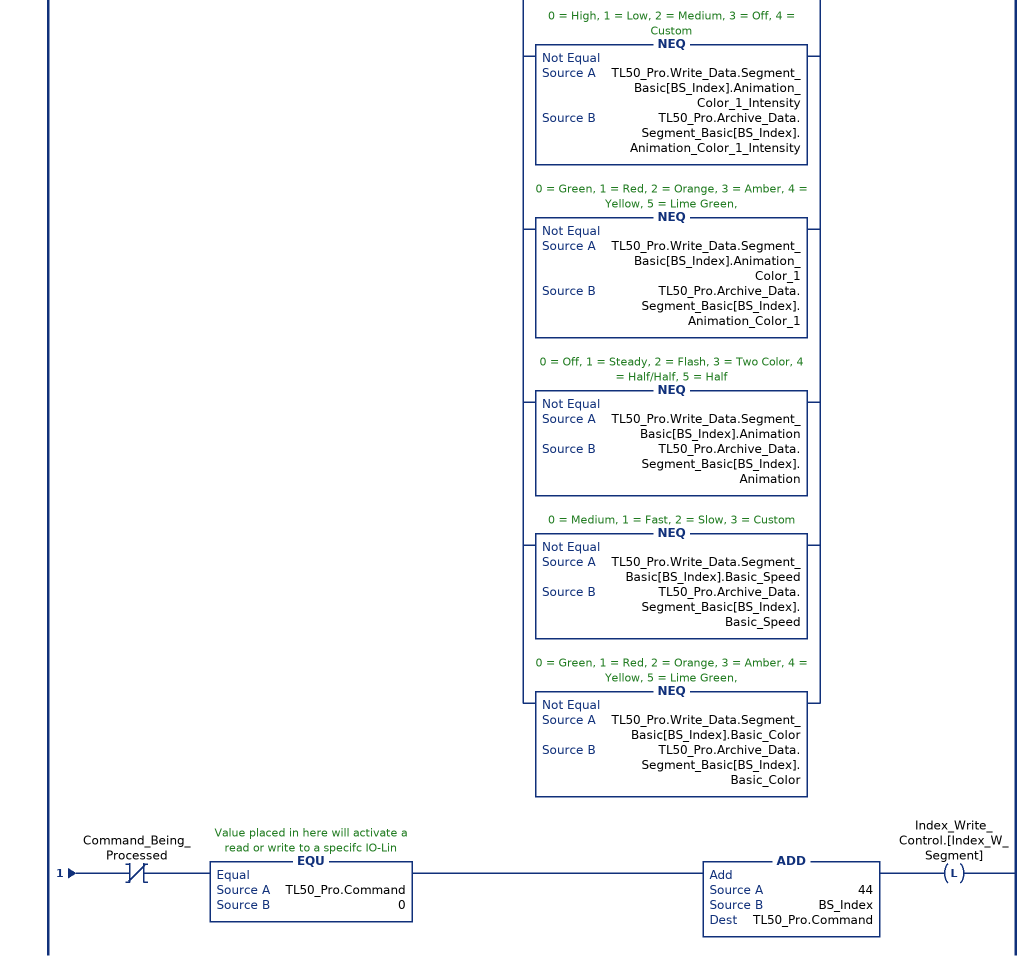
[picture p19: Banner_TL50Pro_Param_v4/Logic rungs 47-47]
   47: XIC(TL50_Pro.Initial_Global_Read)XIO(Local_Control.0)XIO(Index_Write_Control.[Index_W_Segment])XIO(Update_Archive)[NEQ(TL50_Pro.Write_Data.Segment_Basic[BS_Index].Animation_Rotational_Direction,TL50_Pro.Archive_Data.Segment_Basic[BS_Index].Animation_Rotational_Direction) ,NEQ(TL50_Pro.Write_Data.Segment_Basic[BS_Index].Animation_Color_2_Intensity,TL50_Pro.Archive_Data.Segment_Basic[BS_Index].Animation_Color_2_Intensity) ,NEQ(TL50_Pro.Write_Data.Segment_Basic[BS_Index].Animation_Color_2,TL50_Pro.Archive_Data.Segment_Basic[BS_Index].Animation_Color_2) ,NEQ(TL50_Pro.Write_Data.Segment_Basic[BS_Index].Animation_Pattern,TL50_Pro.Archive_Data.Segment_Basic[BS_Index].Animation_Pattern) ,NEQ(TL50_Pro.Write_Data.Segment_Basic[BS_Index].Animation_Speed,TL50_Pro.Archive_Data.Segment_Basic[BS_Index].Animation_Speed) ,NEQ(TL50_Pro.Write_Data.Segment_Basic[BS_Index].Animation_Color_1_Intensity,TL50_Pro.Archive_Data.Segment_Basic[BS_Index].Animation_Color_1_Intensity) ,NEQ(TL50_Pro.Write_Data.Segment_Basic[BS_Index].Animation_Color_1,TL50_Pro.Archive_Data.Segment_Basic[BS_Index].Animation_Color_1) ,NEQ(TL50_Pro.Write_Data.Segment_Basic[BS_Index].Animation,TL50_Pro.Archive_Data.Segment_Basic[BS_Index].Animation) ,NEQ(TL50_Pro.Write_Data.Segment_Basic[BS_Index].Basic_Speed,TL50_Pro.Archive_Data.Segment_Basic[BS_Index].Basic_Speed) ,NEQ(TL50_Pro.Write_Data.Segment_Basic[BS_Index].Basic_Color,TL50_Pro.Archive_Data.Segment_Basic[BS_Index].Basic_Color) ]OTL(Index_Write_Inprocess.[Index_W_Segment])XIO(Command_Being_Processed)EQU(TL50_Pro.Command,0)ADD(44,BS_Index,TL50_Pro.Command)OTL(Index_Write_Control.[Index_W_Segment]);
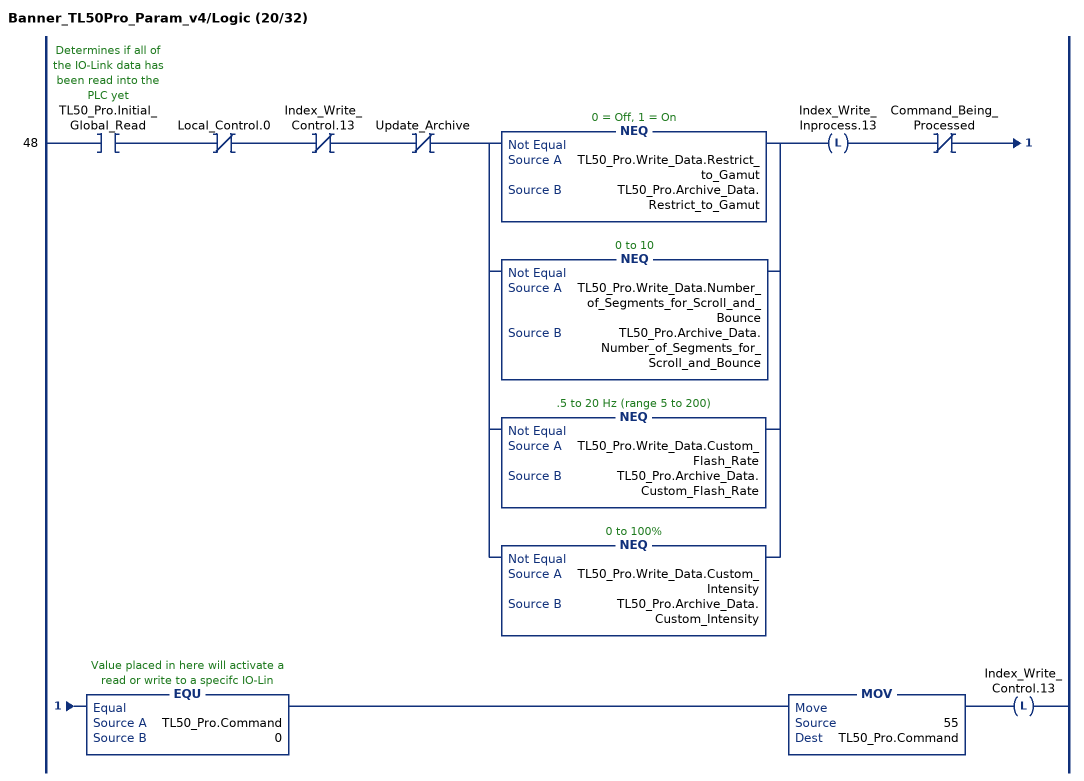
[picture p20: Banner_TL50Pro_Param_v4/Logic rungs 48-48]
   48: XIC(TL50_Pro.Initial_Global_Read)XIO(Local_Control.0)XIO(Index_Write_Control.13)XIO(Update_Archive)[NEQ(TL50_Pro.Write_Data.Restrict_to_Gamut,TL50_Pro.Archive_Data.Restrict_to_Gamut) ,NEQ(TL50_Pro.Write_Data.Number_of_Segments_for_Scroll_and_Bounce,TL50_Pro.Archive_Data.Number_of_Segments_for_Scroll_and_Bounce) ,NEQ(TL50_Pro.Write_Data.Custom_Flash_Rate,TL50_Pro.Archive_Data.Custom_Flash_Rate) ,NEQ(TL50_Pro.Write_Data.Custom_Intensity,TL50_Pro.Archive_Data.Custom_Intensity) ]OTL(Index_Write_Inprocess.13)XIO(Command_Being_Processed)EQU(TL50_Pro.Command,0)MOV(55,TL50_Pro.Command)OTL(Index_Write_Control.13);
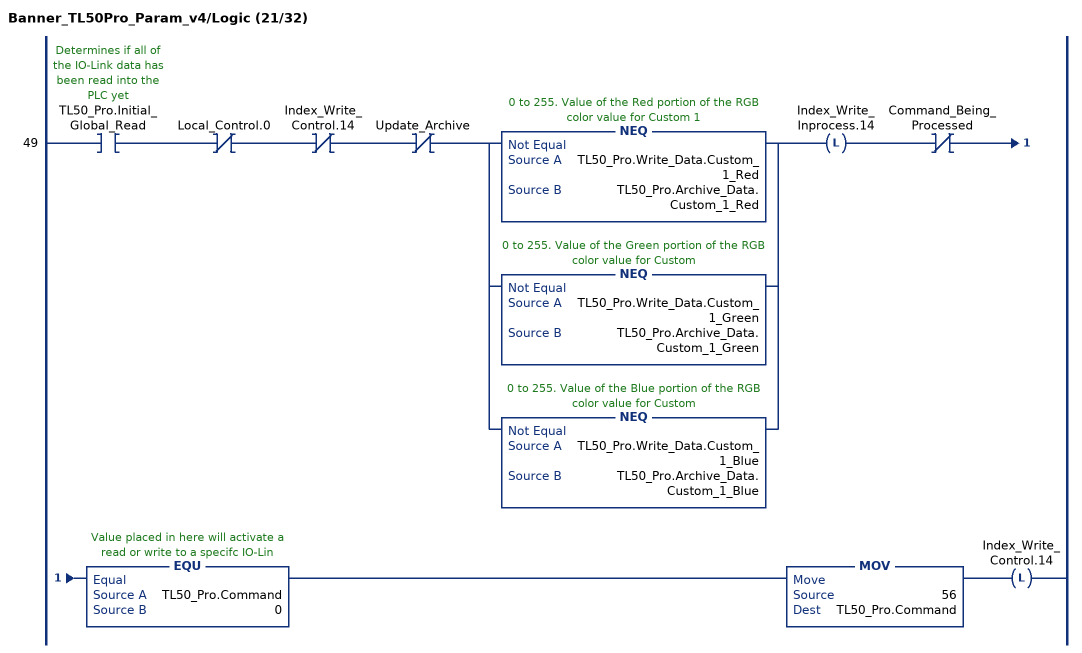
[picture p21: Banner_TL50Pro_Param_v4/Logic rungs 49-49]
   49: XIC(TL50_Pro.Initial_Global_Read)XIO(Local_Control.0)XIO(Index_Write_Control.14)XIO(Update_Archive)[NEQ(TL50_Pro.Write_Data.Custom_1_Red,TL50_Pro.Archive_Data.Custom_1_Red) ,NEQ(TL50_Pro.Write_Data.Custom_1_Green,TL50_Pro.Archive_Data.Custom_1_Green) ,NEQ(TL50_Pro.Write_Data.Custom_1_Blue,TL50_Pro.Archive_Data.Custom_1_Blue) ]OTL(Index_Write_Inprocess.14)XIO(Command_Being_Processed)EQU(TL50_Pro.Command,0)MOV(56,TL50_Pro.Command)OTL(Index_Write_Control.14);
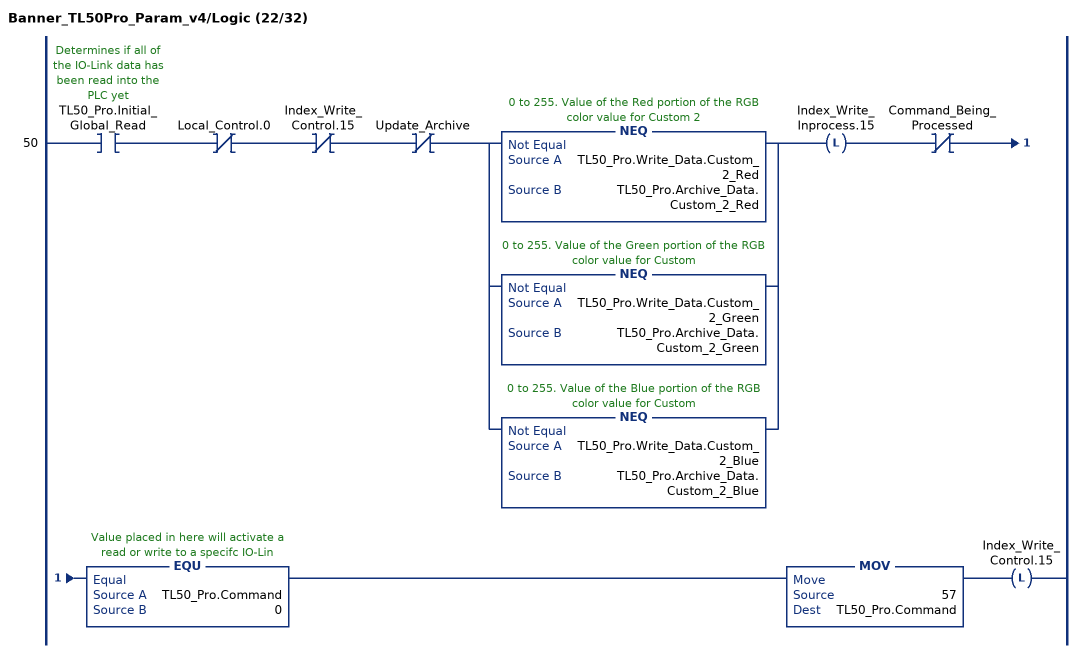
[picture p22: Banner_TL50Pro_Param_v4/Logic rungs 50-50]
   50: XIC(TL50_Pro.Initial_Global_Read)XIO(Local_Control.0)XIO(Index_Write_Control.15)XIO(Update_Archive)[NEQ(TL50_Pro.Write_Data.Custom_2_Red,TL50_Pro.Archive_Data.Custom_2_Red) ,NEQ(TL50_Pro.Write_Data.Custom_2_Green,TL50_Pro.Archive_Data.Custom_2_Green) ,NEQ(TL50_Pro.Write_Data.Custom_2_Blue,TL50_Pro.Archive_Data.Custom_2_Blue) ]OTL(Index_Write_Inprocess.15)XIO(Command_Being_Processed)EQU(TL50_Pro.Command,0)MOV(57,TL50_Pro.Command)OTL(Index_Write_Control.15);
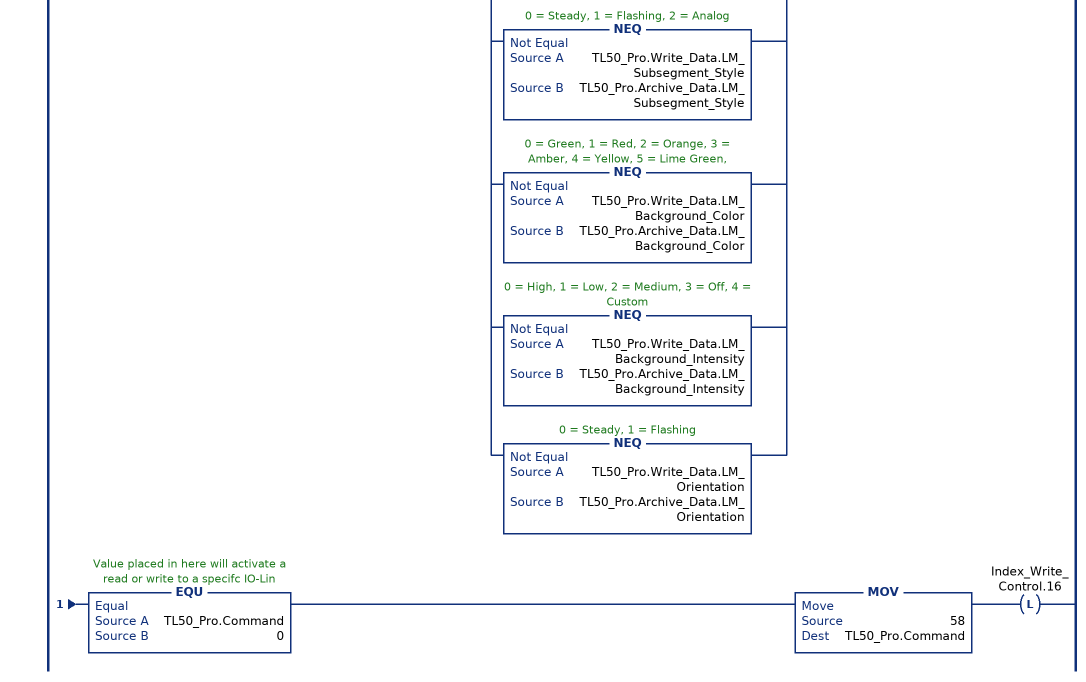
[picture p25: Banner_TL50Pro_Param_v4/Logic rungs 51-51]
   51: XIC(TL50_Pro.Initial_Global_Read)XIO(Local_Control.0)XIO(Index_Write_Control.16)XIO(Update_Archive)[NEQ(TL50_Pro.Write_Data.LM_Full_Scale_Value,TL50_Pro.Archive_Data.LM_Full_Scale_Value) ,NEQ(TL50_Pro.Write_Data.LM_Base_Color,TL50_Pro.Archive_Data.LM_Base_Color) ,NEQ(TL50_Pro.Write_Data.LM_Base_Intensity,TL50_Pro.Archive_Data.LM_Base_Intensity) ,NEQ(TL50_Pro.Write_Data.LM_Base_State,TL50_Pro.Archive_Data.LM_Base_State) ,NEQ(TL50_Pro.Write_Data.LM_Threshold_Type,TL50_Pro.Archive_Data.LM_Threshold_Type) ,NEQ(TL50_Pro.Write_Data.LM_Low_Threshold_Value,TL50_Pro.Archive_Data.LM_Low_Threshold_Value) ,NEQ(TL50_Pro.Write_Data.LM_Low_Threshold_Color,TL50_Pro.Archive_Data.LM_Low_Threshold_Color) ,NEQ(TL50_Pro.Write_Data.LM_Low_Threshold_Intensity,TL50_Pro.Archive_Data.LM_Low_Threshold_Intensity) ,NEQ(TL50_Pro.Write_Data.LM_Low_Threshold_State,TL50_Pro.Archive_Data.LM_Low_Threshold_State) ,NEQ(TL50_Pro.Write_Data.LM_High_Threshold_Value,TL50_Pro.Archive_Data.LM_High_Threshold_Value) ,NEQ(TL50_Pro.Write_Data.LM_High_Threshold_Color,TL50_Pro.Archive_Data.LM_High_Threshold_Color) ,NEQ(TL50_Pro.Write_Data.LM_High_Threshold_Intensity,TL50_Pro.Archive_Data.LM_High_Threshold_Intensity) ,NEQ(TL50_Pro.Write_Data.LM_High_Threshold_State,TL50_Pro.Archive_Data.LM_High_Threshold_State) ,NEQ(TL50_Pro.Write_Data.LM_Flash_Rate,TL50_Pro.Archive_Data.LM_Flash_Rate) ,NEQ(TL50_Pro.Write_Data.LM_Dominance,TL50_Pro.Archive_Data.LM_Dominance) ,NEQ(TL50_Pro.Write_Data.LM_Subsegment_Style,TL50_Pro.Archive_Data.LM_Subsegment_Style) ,NEQ(TL50_Pro.Write_Data.LM_Background_Color,TL50_Pro.Archive_Data.LM_Background_Color) ,NEQ(TL50_Pro.Write_Data.LM_Background_Intensity,TL50_Pro.Archive_Data.LM_Background_Intensity) ,NEQ(TL50_Pro.Write_Data.LM_Orientation,TL50_Pro.Archive_Data.LM_Orientation) ]OTL(Index_Write_Inprocess.16)XIO(Command_Being_Processed)EQU(TL50_Pro.Command,0)MOV(58,TL50_Pro.Command)OTL(Index_Write_Control.16);
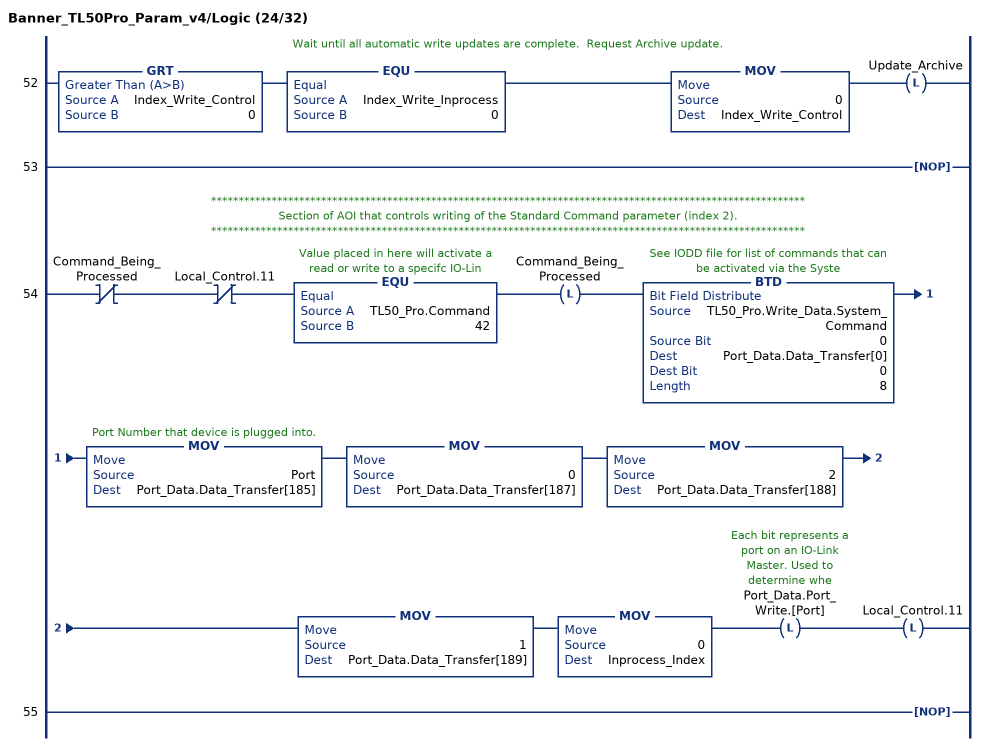
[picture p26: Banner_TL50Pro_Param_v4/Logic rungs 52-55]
   // Wait until all automatic write updates are complete.  Request Archive update.
   52: GRT(Index_Write_Control,0)EQU(Index_Write_Inprocess,0)MOV(0,Index_Write_Control)OTL(Update_Archive);
   53: NOP();
   // ************************************************************************************************************
   // Section of AOI that controls writing of the Standard Command parameter (index 2).
   // ************************************************************************************************************
   54: XIO(Command_Being_Processed)XIO(Local_Control.11)EQU(TL50_Pro.Command,42)OTL(Command_Being_Processed)BTD(TL50_Pro.Write_Data.System_Command,0,Port_Data.Data_Transfer[0],0,8)MOV(Port,Port_Data.Data_Transfer[185])MOV(0,Port_Data.Data_Transfer[187])MOV(2,Port_Data.Data_Transfer[188])MOV(1,Port_Data.Data_Transfer[189])MOV(0,Inprocess_Index)OTL(Port_Data.Port_Write.[Port])OTL(Local_Control.11);
   55: NOP();
